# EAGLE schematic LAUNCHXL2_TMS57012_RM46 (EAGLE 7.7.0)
DOC_NUMBER: LAUNCHXL2_TMS57012_RM46; REV: B

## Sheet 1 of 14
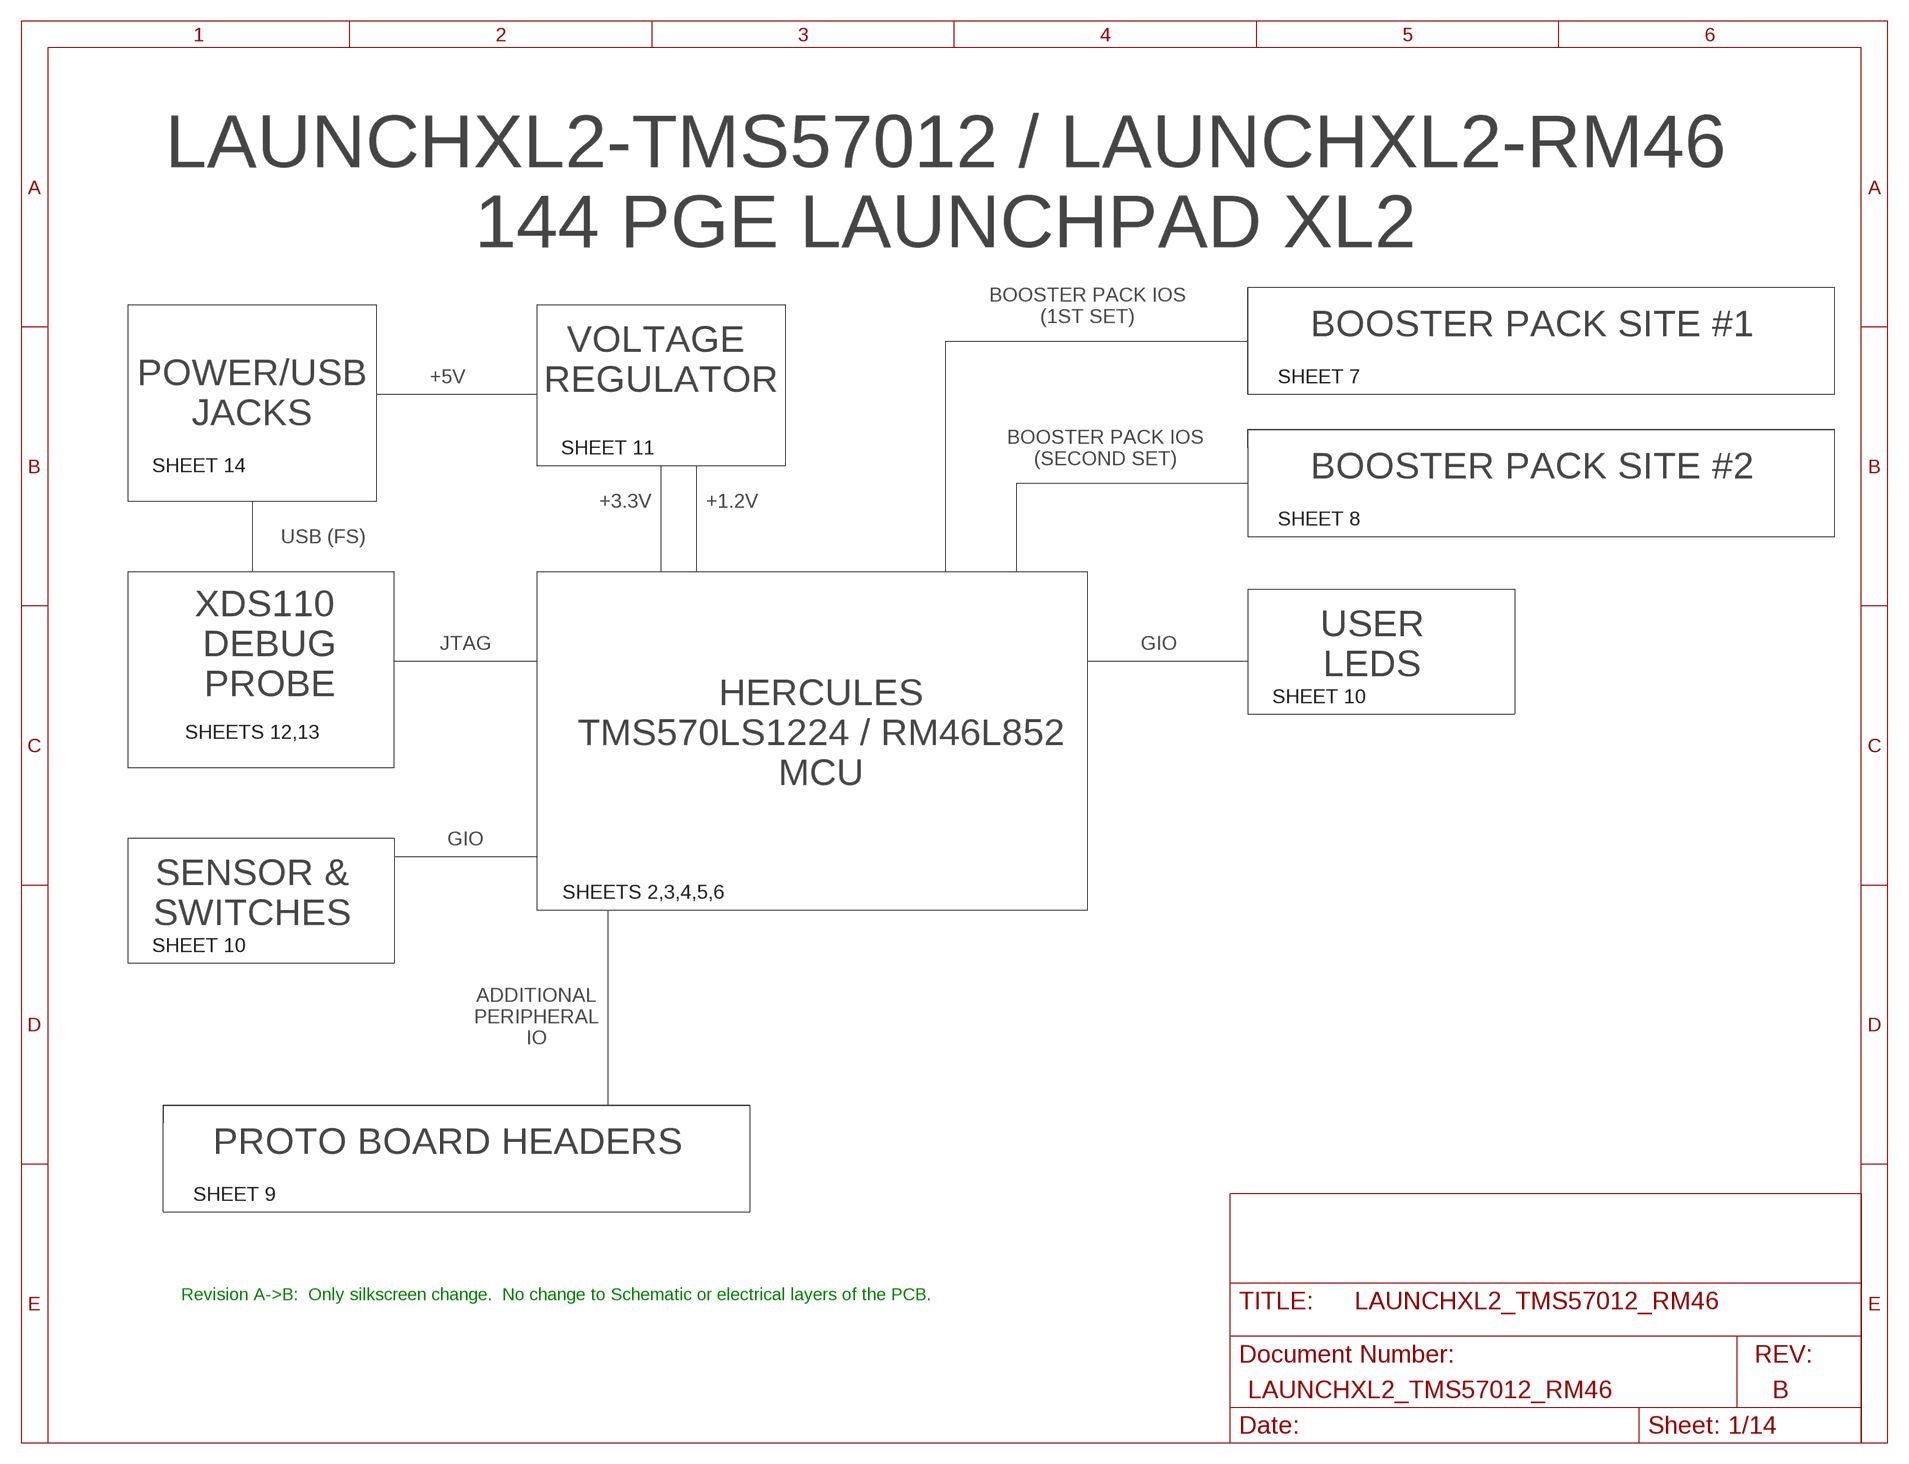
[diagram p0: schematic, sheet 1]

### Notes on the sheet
- LAUNCHXL2-TMS57012 / LAUNCHXL2-RM46
  144 PGE LAUNCHPAD XL2
- BOOSTER PACK IOS
  (1ST SET)
- BOOSTER PACK SITE #1
- VOLTAGE 
  REGULATOR
- +5V | SHEET 7
- POWER/USB
  JACKS
- SHEET 11
- BOOSTER PACK IOS
  (SECOND SET)
- SHEET 14 | BOOSTER PACK SITE #2
- +3.3V | +1.2V
- SHEET 8
- USB (FS)
- XDS110 
  DEBUG
  PROBE
- JTAG | GIO
- USER
  LEDS
- SHEET 10
- SHEETS 12,13
- HERCULES
  TMS570LS1224 / RM46L852
  MCU
- GIO
- SENSOR &
  SWITCHES
- SHEETS 2,3,4,5,6
- SHEET 10
- ADDITIONAL
  PERIPHERAL
  IO
- PROTO BOARD HEADERS
- SHEET 9
- Revision A->B:  Only silkscreen change.  No change to Schematic or electrical layers of the PCB.

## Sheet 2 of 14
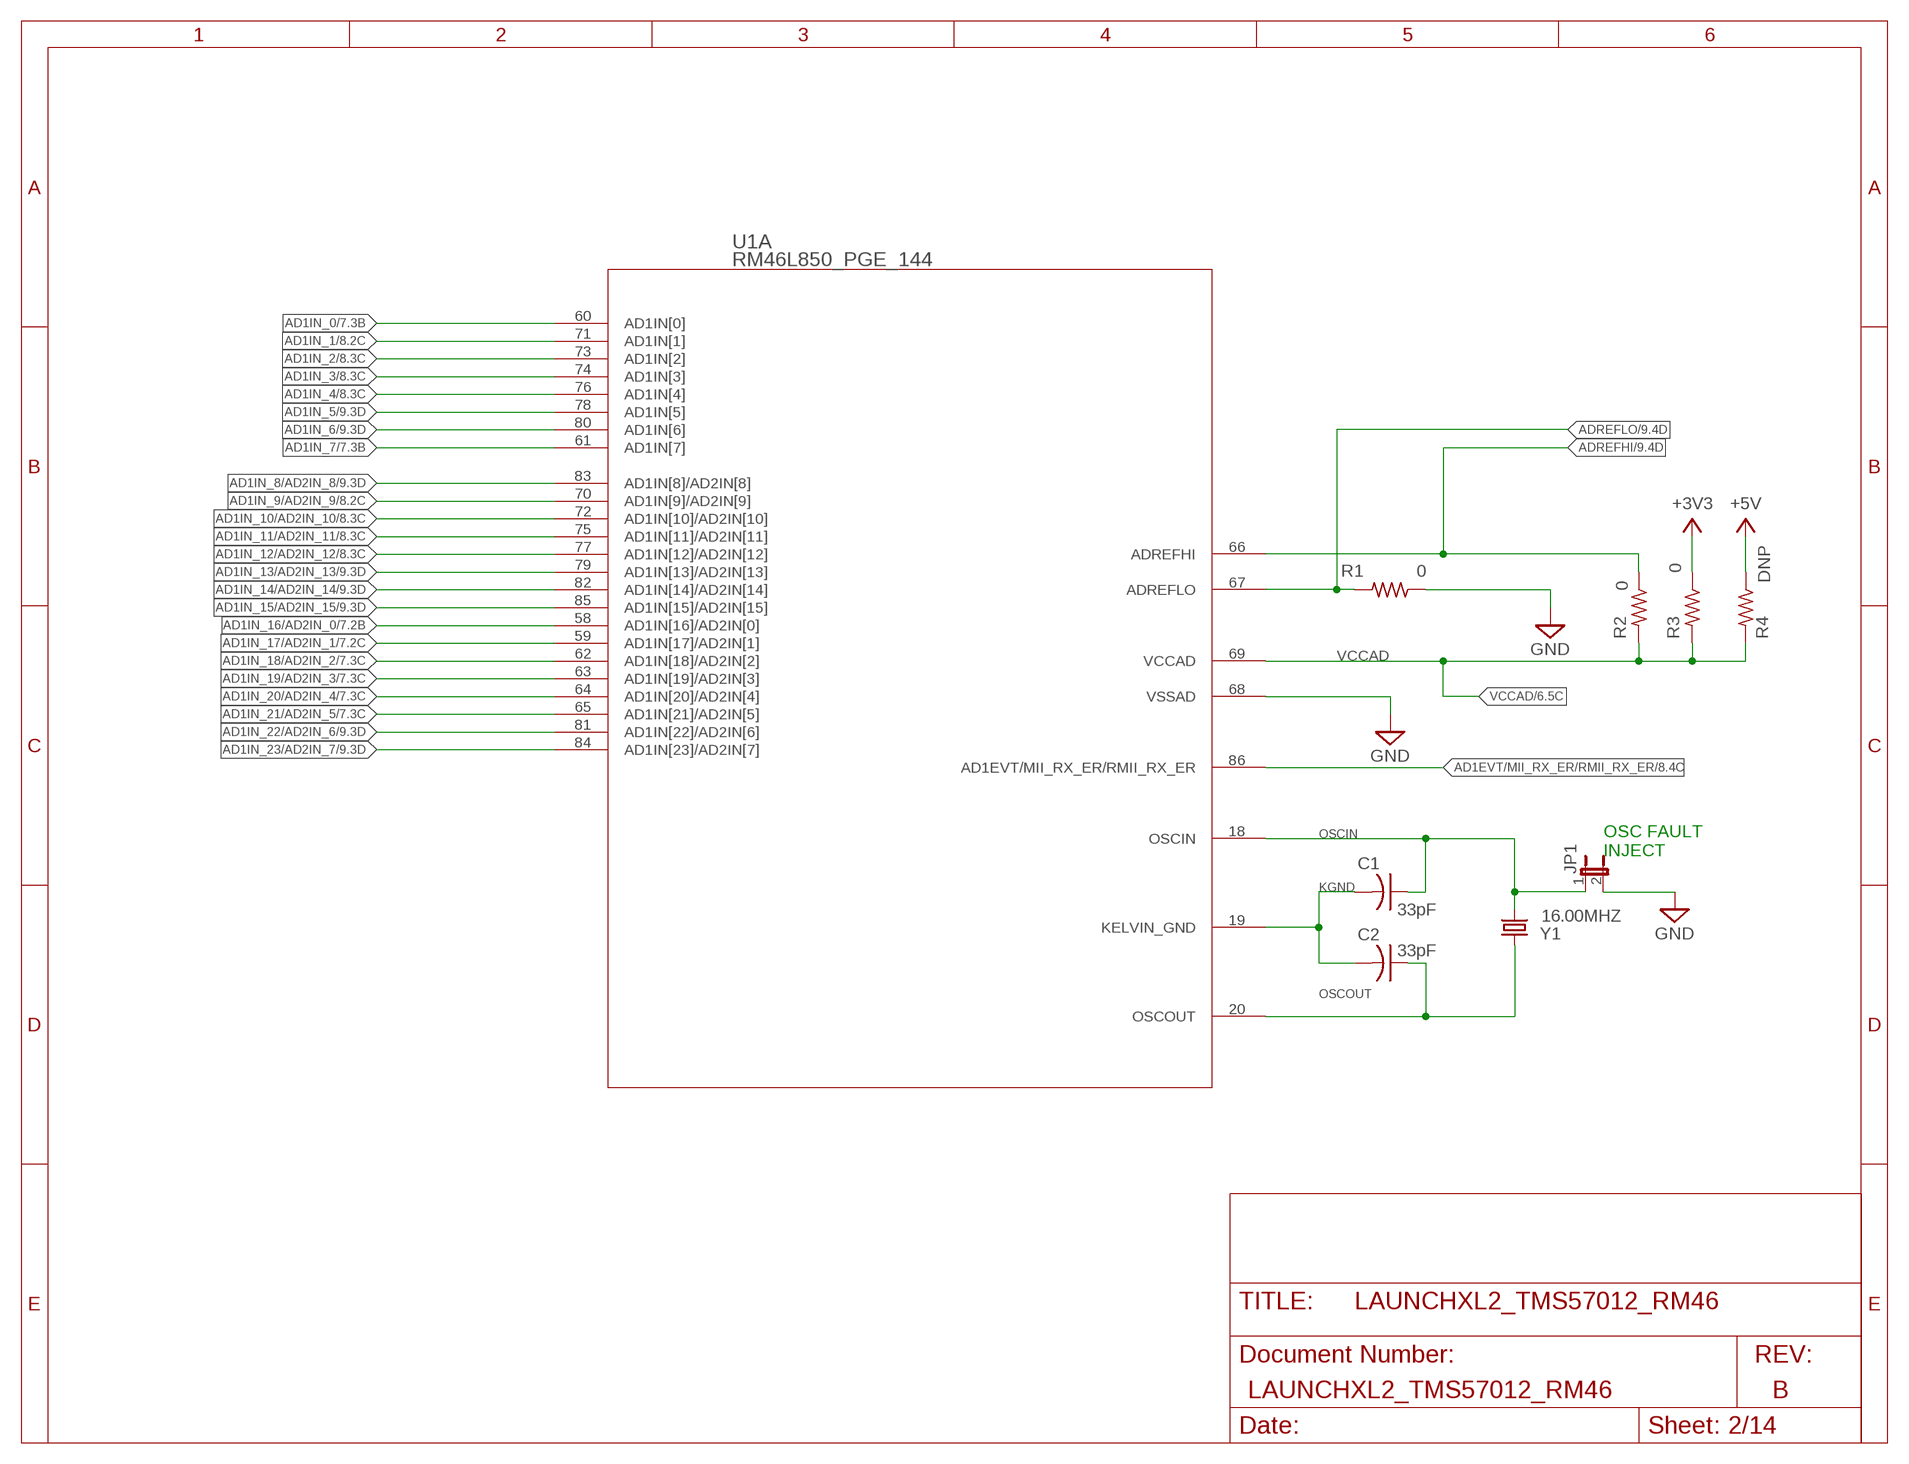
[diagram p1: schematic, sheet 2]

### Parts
C1  33pF  C-USC0402K  [C0402K]
C2  33pF  C-USC0402K  [C0402K]
JP1  SHUNT_HANG_OFF  JP1E  [JP1]
R1  0  R-US_R0402  [R0402]
R2  0  R-US_R0402  [R0402]
R3  0  R-US_R0402  [R0402]
R4  DNP  R-US_R0402  [R0402]
U1  RM46L850_PGE_144  [PGE144]
Y1  16.00MHZ  CRYSTAL  [ABLS]

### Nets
+3V3: R3.1 ; also sheet 3,5,6,7,8,9,10,11,12,13
+5V: R4.1 ; also sheet 7,8,9,11,14
AD1EVT/MII_RX_ER/RMII_RX_ER: U1.86(A:AD1EVT/MII_RX_ER/RMII_RX_ER) ; also sheet 8,9
AD1IN_0: U1.60(A:AD1IN[0]) ; also sheet 7
AD1IN_1: U1.71(A:AD1IN[1]) ; also sheet 8
AD1IN_2: U1.73(A:AD1IN[2]) ; also sheet 8
AD1IN_3: U1.74(A:AD1IN[3]) ; also sheet 8
AD1IN_4: U1.76(A:AD1IN[4]) ; also sheet 8
AD1IN_5: U1.78(A:AD1IN[5]) ; also sheet 9
AD1IN_6: U1.80(A:AD1IN[6]) ; also sheet 9,10
AD1IN_7: U1.61(A:AD1IN[7]) ; also sheet 7
AD1IN_8/AD2IN_8: U1.83(A:AD1IN[8]/AD2IN[8]) ; also sheet 9
AD1IN_9/AD2IN_9: U1.70(A:AD1IN[9]/AD2IN[9]) ; also sheet 8,9
AD1IN_10/AD2IN_10: U1.72(A:AD1IN[10]/AD2IN[10]) ; also sheet 8,9
AD1IN_11/AD2IN_11: U1.75(A:AD1IN[11]/AD2IN[11]) ; also sheet 8,9
AD1IN_12/AD2IN_12: U1.77(A:AD1IN[12]/AD2IN[12]) ; also sheet 8,9
AD1IN_13/AD2IN_13: U1.79(A:AD1IN[13]/AD2IN[13]) ; also sheet 9
AD1IN_14/AD2IN_14: U1.82(A:AD1IN[14]/AD2IN[14]) ; also sheet 9
AD1IN_15/AD2IN_15: U1.85(A:AD1IN[15]/AD2IN[15]) ; also sheet 9
AD1IN_16/AD2IN_0: U1.58(A:AD1IN[16]/AD2IN[0]) ; also sheet 7,9
AD1IN_17/AD2IN_1: U1.59(A:AD1IN[17]/AD2IN[1]) ; also sheet 7,9
AD1IN_18/AD2IN_2: U1.62(A:AD1IN[18]/AD2IN[2]) ; also sheet 7,9
AD1IN_19/AD2IN_3: U1.63(A:AD1IN[19]/AD2IN[3]) ; also sheet 7,9
AD1IN_20/AD2IN_4: U1.64(A:AD1IN[20]/AD2IN[4]) ; also sheet 7,9
AD1IN_21/AD2IN_5: U1.65(A:AD1IN[21]/AD2IN[5]) ; also sheet 7,9
AD1IN_22/AD2IN_6: U1.81(A:AD1IN[22]/AD2IN[6]) ; also sheet 9
AD1IN_23/AD2IN_7: U1.84(A:AD1IN[23]/AD2IN[7]) ; also sheet 9
ADREFHI: R2.1 U1.66(A:ADREFHI) ; also sheet 9
ADREFLO: R1.2 U1.67(A:ADREFLO) ; also sheet 9
GND: JP1.2 R1.1 U1.68(A:VSSAD) ; also sheet 3,5,6,7,8,9,10,11,12,13,14
KGND: C1.2 C2.2 U1.19(A:KELVIN_GND)
OSCIN: C1.1 JP1.1 U1.18(A:OSCIN) Y1.2
OSCOUT: C2.1 U1.20(A:OSCOUT) Y1.1
VCCAD: R2.2 R3.2 R4.2 U1.69(A:VCCAD) ; also sheet 6

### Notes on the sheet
- OSC FAULT
  INJECT

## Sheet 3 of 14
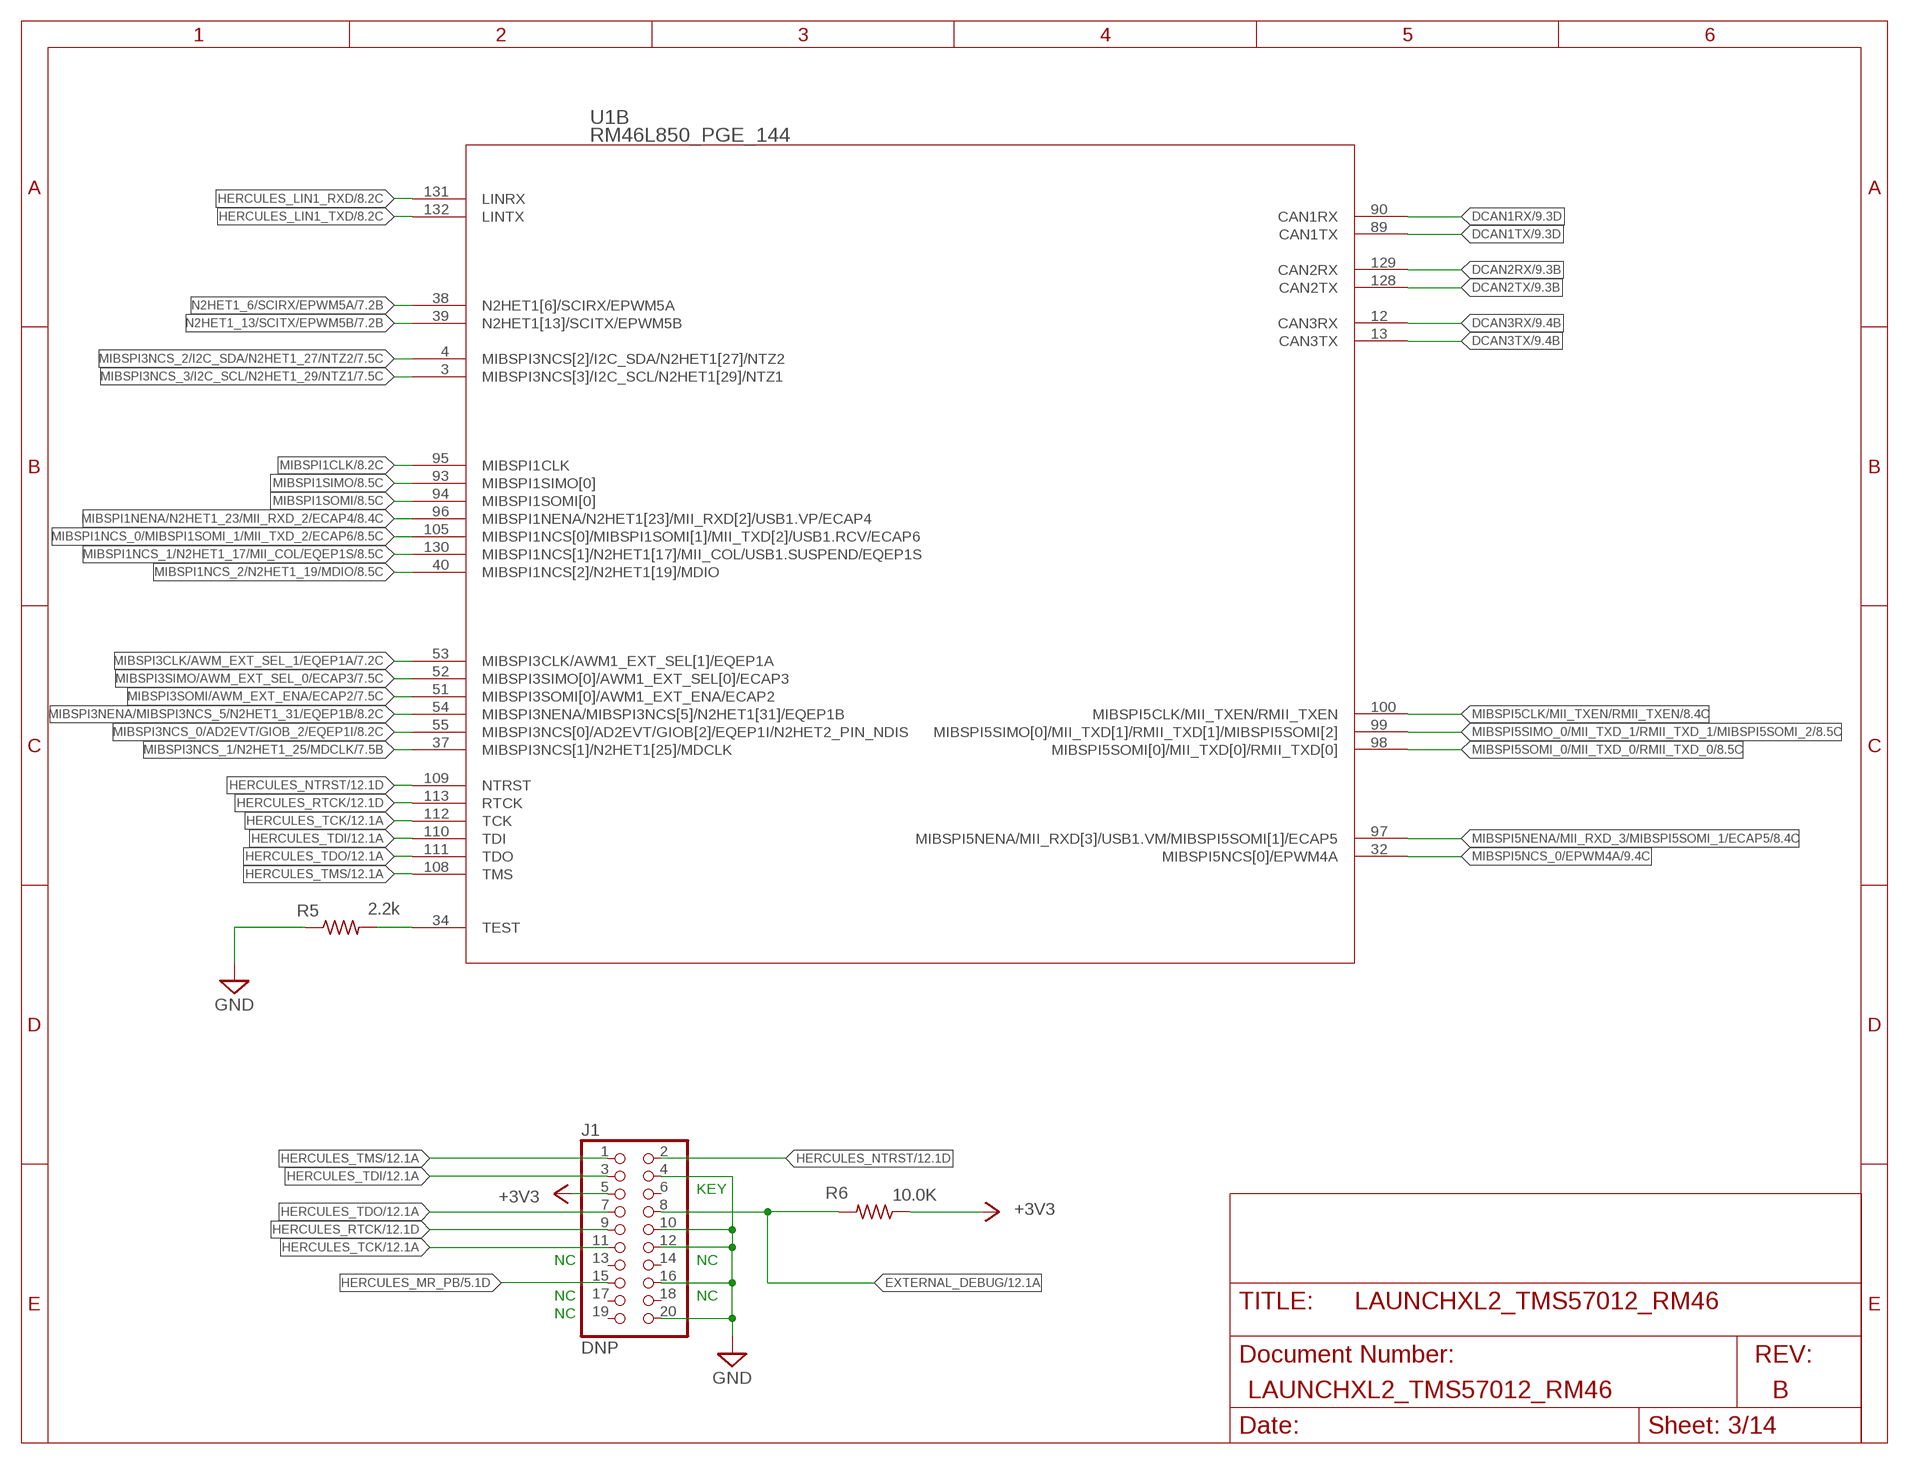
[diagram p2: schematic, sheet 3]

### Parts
J1  DNP  PINHD-2X10SAMTEC-FTR-110-51-S-D-06  [SAMTEC-FTR-110-51-S-D-06]
R5  2.2k  R-US_R0402  [R0402]
R6  10.0K  R-US_R0402  [R0402]

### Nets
+3V3: J1.5 R6.1 ; also sheet 2,5,6,7,8,9,10,11,12,13
DCAN1RX: U1.90(B:CAN1RX) ; also sheet 9
DCAN1TX: U1.89(B:CAN1TX) ; also sheet 9
DCAN2RX: U1.129(B:CAN2RX) ; also sheet 9
DCAN2TX: U1.128(B:CAN2TX) ; also sheet 9
DCAN3RX: U1.12(B:CAN3RX) ; also sheet 9
DCAN3TX: U1.13(B:CAN3TX) ; also sheet 9
EXTERNAL_DEBUG: J1.8 R6.2 ; also sheet 12
GND: J1.4 J1.10 J1.12 J1.16 J1.20 R5.1 ; also sheet 2,5,6,7,8,9,10,11,12,13,14
HERCULES_LIN1_RXD: U1.131(B:LINRX) ; also sheet 8,9,12
HERCULES_LIN1_TXD: U1.132(B:LINTX) ; also sheet 8,9,12
HERCULES_MR_PB: J1.15 ; also sheet 5,12
HERCULES_NTRST: J1.2 U1.109(B:NTRST) ; also sheet 12
HERCULES_RTCK: J1.9 U1.113(B:RTCK) ; also sheet 12
HERCULES_TCK: J1.11 U1.112(B:TCK) ; also sheet 12
HERCULES_TDI: J1.3 U1.110(B:TDI) ; also sheet 12
HERCULES_TDO: J1.7 U1.111(B:TDO) ; also sheet 12
HERCULES_TMS: J1.1 U1.108(B:TMS) ; also sheet 12
MIBSPI1CLK: U1.95(B:MIBSPI1CLK) ; also sheet 8,9
MIBSPI1NCS_0/MIBSPI1SOMI_1/MII_TXD_2/ECAP6: U1.105(B:MIBSPI1NCS[0]/MIBSPI1SOMI[1]/MII_TXD[2]/USB1.RCV/ECAP6) ; also sheet 8,9
MIBSPI1NCS_1/N2HET1_17/MII_COL/EQEP1S: U1.130(B:MIBSPI1NCS[1]/N2HET1[17]/MII_COL/USB1.SUSPEND/EQEP1S) ; also sheet 8,9
MIBSPI1NCS_2/N2HET1_19/MDIO: U1.40(B:MIBSPI1NCS[2]/N2HET1[19]/MDIO) ; also sheet 8,9
MIBSPI1NENA/N2HET1_23/MII_RXD_2/ECAP4: U1.96(B:MIBSPI1NENA/N2HET1[23]/MII_RXD[2]/USB1.VP/ECAP4) ; also sheet 8,9
MIBSPI1SIMO: U1.93(B:MIBSPI1SIMO[0]) ; also sheet 8,9
MIBSPI1SOMI: U1.94(B:MIBSPI1SOMI[0]) ; also sheet 8,9
MIBSPI3CLK/AWM_EXT_SEL_1/EQEP1A: U1.53(B:MIBSPI3CLK/AWM1_EXT_SEL[1]/EQEP1A) ; also sheet 7,9
MIBSPI3NCS_0/AD2EVT/GIOB_2/EQEP1I: U1.55(B:MIBSPI3NCS[0]/AD2EVT/GIOB[2]/EQEP1I/N2HET2_PIN_NDIS) ; also sheet 8,9,10
MIBSPI3NCS_1/N2HET1_25/MDCLK: U1.37(B:MIBSPI3NCS[1]/N2HET1[25]/MDCLK) ; also sheet 7,9
MIBSPI3NCS_2/I2C_SDA/N2HET1_27/NTZ2: U1.4(B:MIBSPI3NCS[2]/I2C_SDA/N2HET1[27]/NTZ2) ; also sheet 7,9
MIBSPI3NCS_3/I2C_SCL/N2HET1_29/NTZ1: U1.3(B:MIBSPI3NCS[3]/I2C_SCL/N2HET1[29]/NTZ1) ; also sheet 7,9
MIBSPI3NENA/MIBSPI3NCS_5/N2HET1_31/EQEP1B: U1.54(B:MIBSPI3NENA/MIBSPI3NCS[5]/N2HET1[31]/EQEP1B) ; also sheet 8,9
MIBSPI3SIMO/AWM_EXT_SEL_0/ECAP3: U1.52(B:MIBSPI3SIMO[0]/AWM1_EXT_SEL[0]/ECAP3) ; also sheet 7,9
MIBSPI3SOMI/AWM_EXT_ENA/ECAP2: U1.51(B:MIBSPI3SOMI[0]/AWM1_EXT_ENA/ECAP2) ; also sheet 7,9
MIBSPI5CLK/MII_TXEN/RMII_TXEN: U1.100(B:MIBSPI5CLK/MII_TXEN/RMII_TXEN) ; also sheet 8,9
MIBSPI5NCS_0/EPWM4A: U1.32(B:MIBSPI5NCS[0]/EPWM4A) ; also sheet 9
MIBSPI5NENA/MII_RXD_3/MIBSPI5SOMI_1/ECAP5: U1.97(B:MIBSPI5NENA/MII_RXD[3]/USB1.VM/MIBSPI5SOMI[1]/ECAP5) ; also sheet 8,9
MIBSPI5SIMO_0/MII_TXD_1/RMII_TXD_1/MIBSPI5SOMI_2: U1.99(B:MIBSPI5SIMO[0]/MII_TXD[1]/RMII_TXD[1]/MIBSPI5SOMI[2]) ; also sheet 8,9
MIBSPI5SOMI_0/MII_TXD_0/RMII_TXD_0: U1.98(B:MIBSPI5SOMI[0]/MII_TXD[0]/RMII_TXD[0]) ; also sheet 8,9
N2HET1_6/SCIRX/EPWM5A: U1.38(B:N2HET1[6]/SCIRX/EPWM5A) ; also sheet 7,9
N2HET1_13/SCITX/EPWM5B: U1.39(B:N2HET1[13]/SCITX/EPWM5B) ; also sheet 7,9
N$39: R5.2 U1.34(B:TEST)
Unconnected: J1.6 J1.13 J1.14 J1.17 J1.18 J1.19

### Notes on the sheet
- KEY
- NC | NC
- NC | NC
- NC

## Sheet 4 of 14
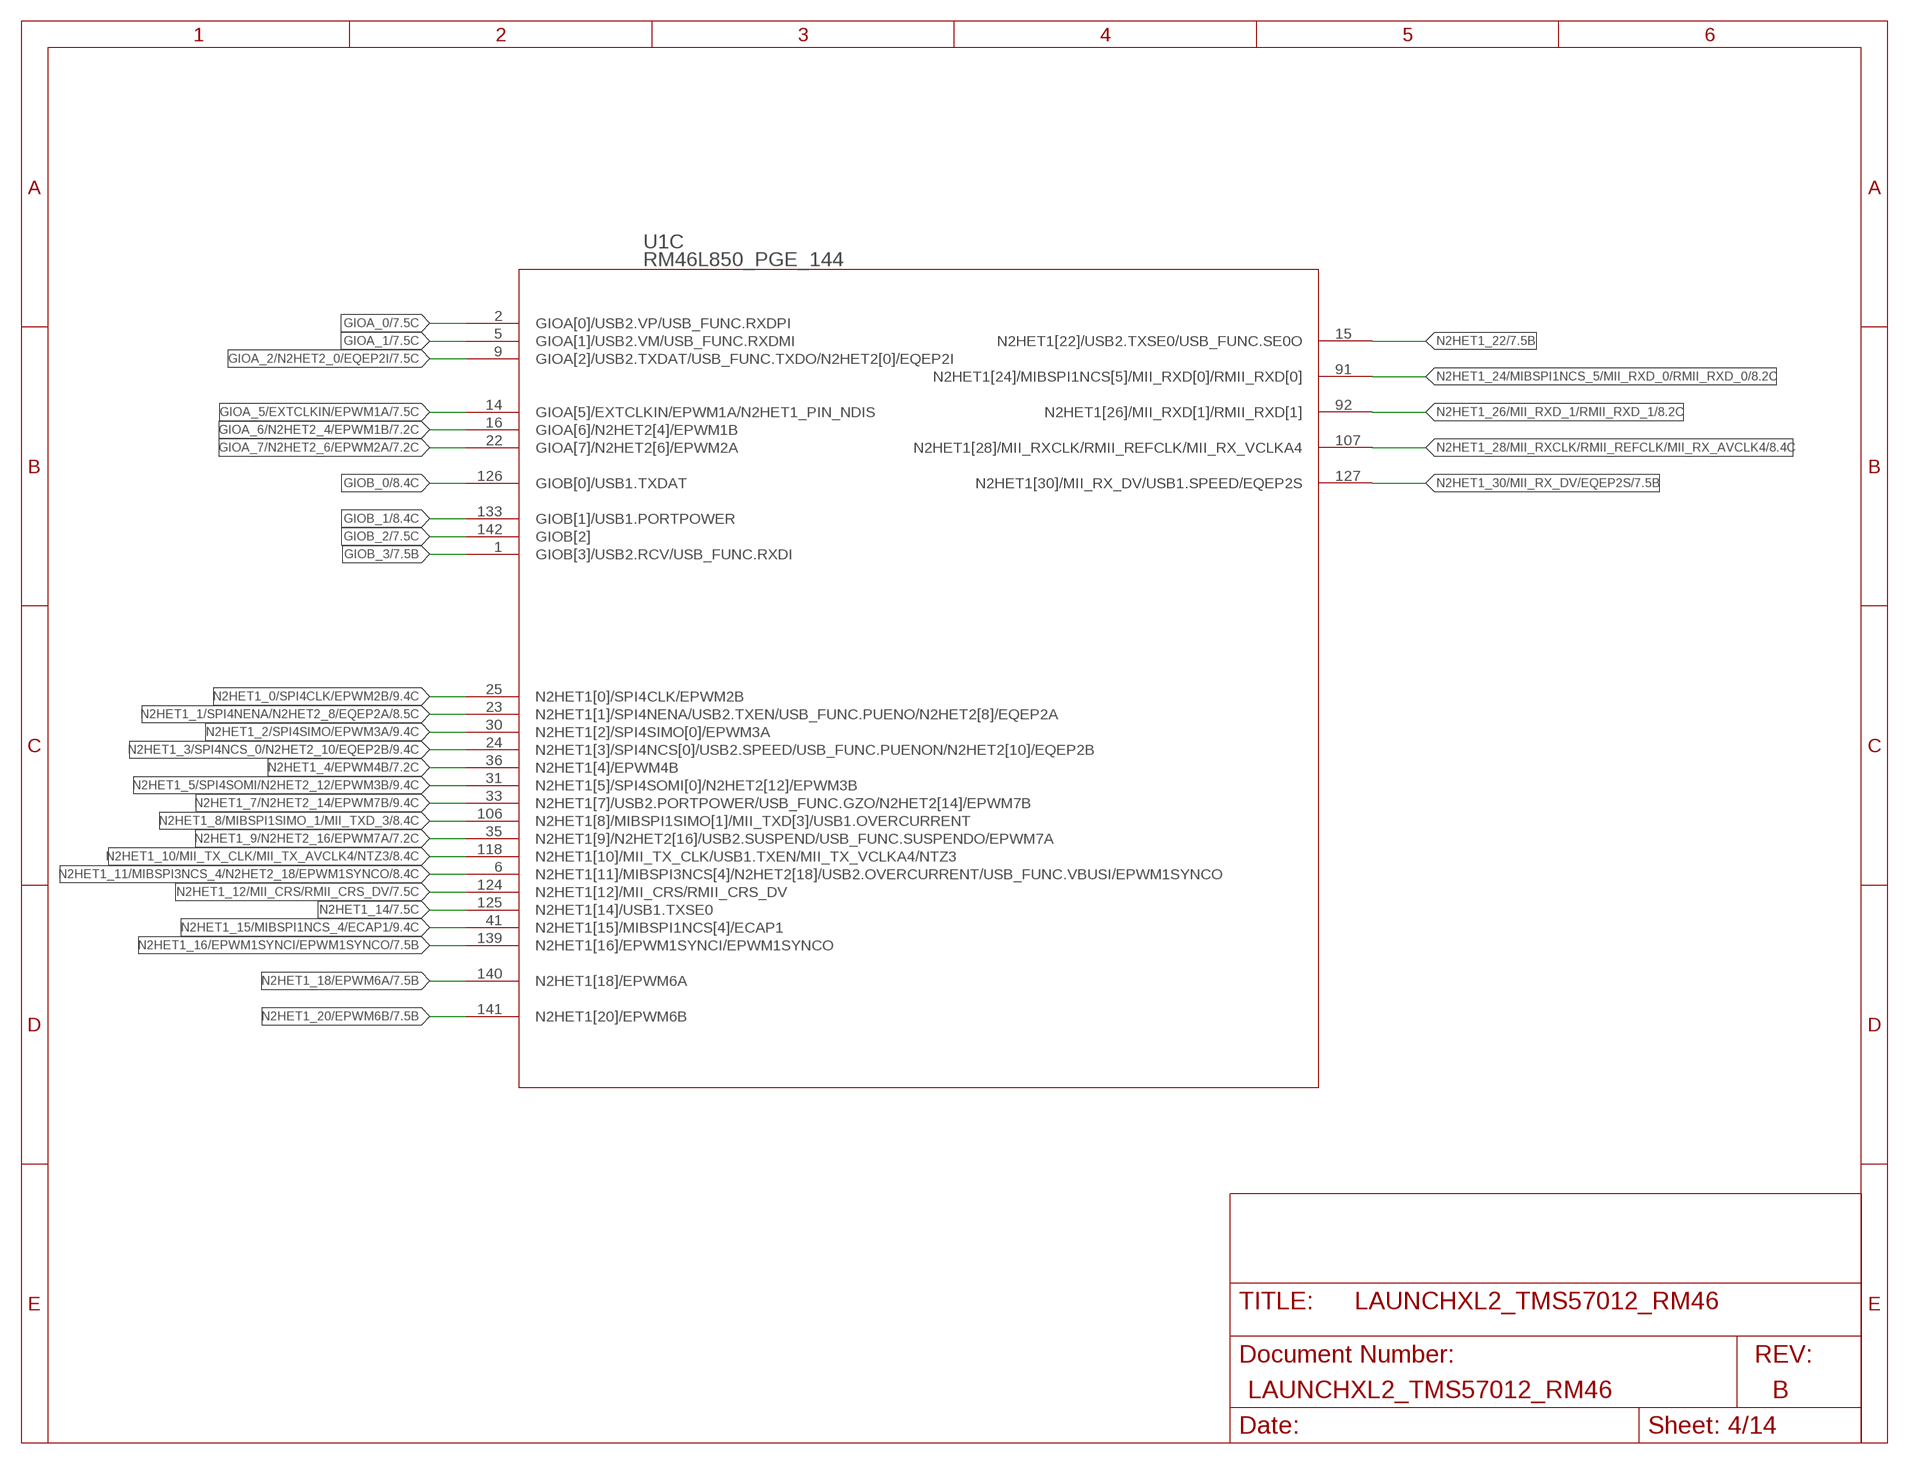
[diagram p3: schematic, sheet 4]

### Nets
GIOA_0: U1.2(C:GIOA[0]/USB2.VP/USB_FUNC.RXDPI) ; also sheet 7,9
GIOA_1: U1.5(C:GIOA[1]/USB2.VM/USB_FUNC.RXDMI) ; also sheet 7,9
GIOA_2/N2HET2_0/EQEP2I: U1.9(C:GIOA[2]/USB2.TXDAT/USB_FUNC.TXDO/N2HET2[0]/EQEP2I) ; also sheet 7,9
GIOA_5/EXTCLKIN/EPWM1A: U1.14(C:GIOA[5]/EXTCLKIN/EPWM1A/N2HET1_PIN_NDIS) ; also sheet 7,9
GIOA_6/N2HET2_4/EPWM1B: U1.16(C:GIOA[6]/N2HET2[4]/EPWM1B) ; also sheet 7,9
GIOA_7/N2HET2_6/EPWM2A: U1.22(C:GIOA[7]/N2HET2[6]/EPWM2A) ; also sheet 7,9
GIOB_0: U1.126(C:GIOB[0]/USB1.TXDAT) ; also sheet 8,9
GIOB_1: U1.133(C:GIOB[1]/USB1.PORTPOWER) ; also sheet 8,9,10
GIOB_2: U1.142(C:GIOB[2]) ; also sheet 7,9,10
GIOB_3: U1.1(C:GIOB[3]/USB2.RCV/USB_FUNC.RXDI) ; also sheet 7,9
N2HET1_0/SPI4CLK/EPWM2B: U1.25(C:N2HET1[0]/SPI4CLK/EPWM2B) ; also sheet 9
N2HET1_1/SPI4NENA/N2HET2_8/EQEP2A: U1.23(C:N2HET1[1]/SPI4NENA/USB2.TXEN/USB_FUNC.PUENO/N2HET2[8]/EQEP2A) ; also sheet 8,9
N2HET1_2/SPI4SIMO/EPWM3A: U1.30(C:N2HET1[2]/SPI4SIMO[0]/EPWM3A) ; also sheet 9
N2HET1_3/SPI4NCS_0/N2HET2_10/EQEP2B: U1.24(C:N2HET1[3]/SPI4NCS[0]/USB2.SPEED/USB_FUNC.PUENON/N2HET2[10]/EQEP2B) ; also sheet 9
N2HET1_4/EPWM4B: U1.36(C:N2HET1[4]/EPWM4B) ; also sheet 7,9
N2HET1_5/SPI4SOMI/N2HET2_12/EPWM3B: U1.31(C:N2HET1[5]/SPI4SOMI[0]/N2HET2[12]/EPWM3B) ; also sheet 9
N2HET1_7/N2HET2_14/EPWM7B: U1.33(C:N2HET1[7]/USB2.PORTPOWER/USB_FUNC.GZO/N2HET2[14]/EPWM7B) ; also sheet 9
N2HET1_8/MIBSPI1SIMO_1/MII_TXD_3: U1.106(C:N2HET1[8]/MIBSPI1SIMO[1]/MII_TXD[3]/USB1.OVERCURRENT) ; also sheet 8,9
N2HET1_9/N2HET2_16/EPWM7A: U1.35(C:N2HET1[9]/N2HET2[16]/USB2.SUSPEND/USB_FUNC.SUSPENDO/EPWM7A) ; also sheet 7,9
N2HET1_10/MII_TX_CLK/MII_TX_AVCLK4/NTZ3: U1.118(C:N2HET1[10]/MII_TX_CLK/USB1.TXEN/MII_TX_VCLKA4/NTZ3) ; also sheet 8,9
N2HET1_11/MIBSPI3NCS_4/N2HET2_18/EPWM1SYNCO: U1.6(C:N2HET1[11]/MIBSPI3NCS[4]/N2HET2[18]/USB2.OVERCURRENT/USB_FUNC.VBUSI/EPWM1SYNCO) ; also sheet 8,9
N2HET1_12/MII_CRS/RMII_CRS_DV: U1.124(C:N2HET1[12]/MII_CRS/RMII_CRS_DV) ; also sheet 7,9
N2HET1_14: U1.125(C:N2HET1[14]/USB1.TXSE0) ; also sheet 7,9
N2HET1_15/MIBSPI1NCS_4/ECAP1: U1.41(C:N2HET1[15]/MIBSPI1NCS[4]/ECAP1) ; also sheet 9,10
N2HET1_16/EPWM1SYNCI/EPWM1SYNCO: U1.139(C:N2HET1[16]/EPWM1SYNCI/EPWM1SYNCO) ; also sheet 7,9
N2HET1_18/EPWM6A: U1.140(C:N2HET1[18]/EPWM6A) ; also sheet 7,9
N2HET1_20/EPWM6B: U1.141(C:N2HET1[20]/EPWM6B) ; also sheet 7,9
N2HET1_22: U1.15(C:N2HET1[22]/USB2.TXSE0/USB_FUNC.SE0O) ; also sheet 7,9
N2HET1_24/MIBSPI1NCS_5/MII_RXD_0/RMII_RXD_0: U1.91(C:N2HET1[24]/MIBSPI1NCS[5]/MII_RXD[0]/RMII_RXD[0]) ; also sheet 8,9
N2HET1_26/MII_RXD_1/RMII_RXD_1: U1.92(C:N2HET1[26]/MII_RXD[1]/RMII_RXD[1]) ; also sheet 8,9
N2HET1_28/MII_RXCLK/RMII_REFCLK/MII_RX_AVCLK4: U1.107(C:N2HET1[28]/MII_RXCLK/RMII_REFCLK/MII_RX_VCLKA4) ; also sheet 8,9
N2HET1_30/MII_RX_DV/EQEP2S: U1.127(C:N2HET1[30]/MII_RX_DV/USB1.SPEED/EQEP2S) ; also sheet 7,9

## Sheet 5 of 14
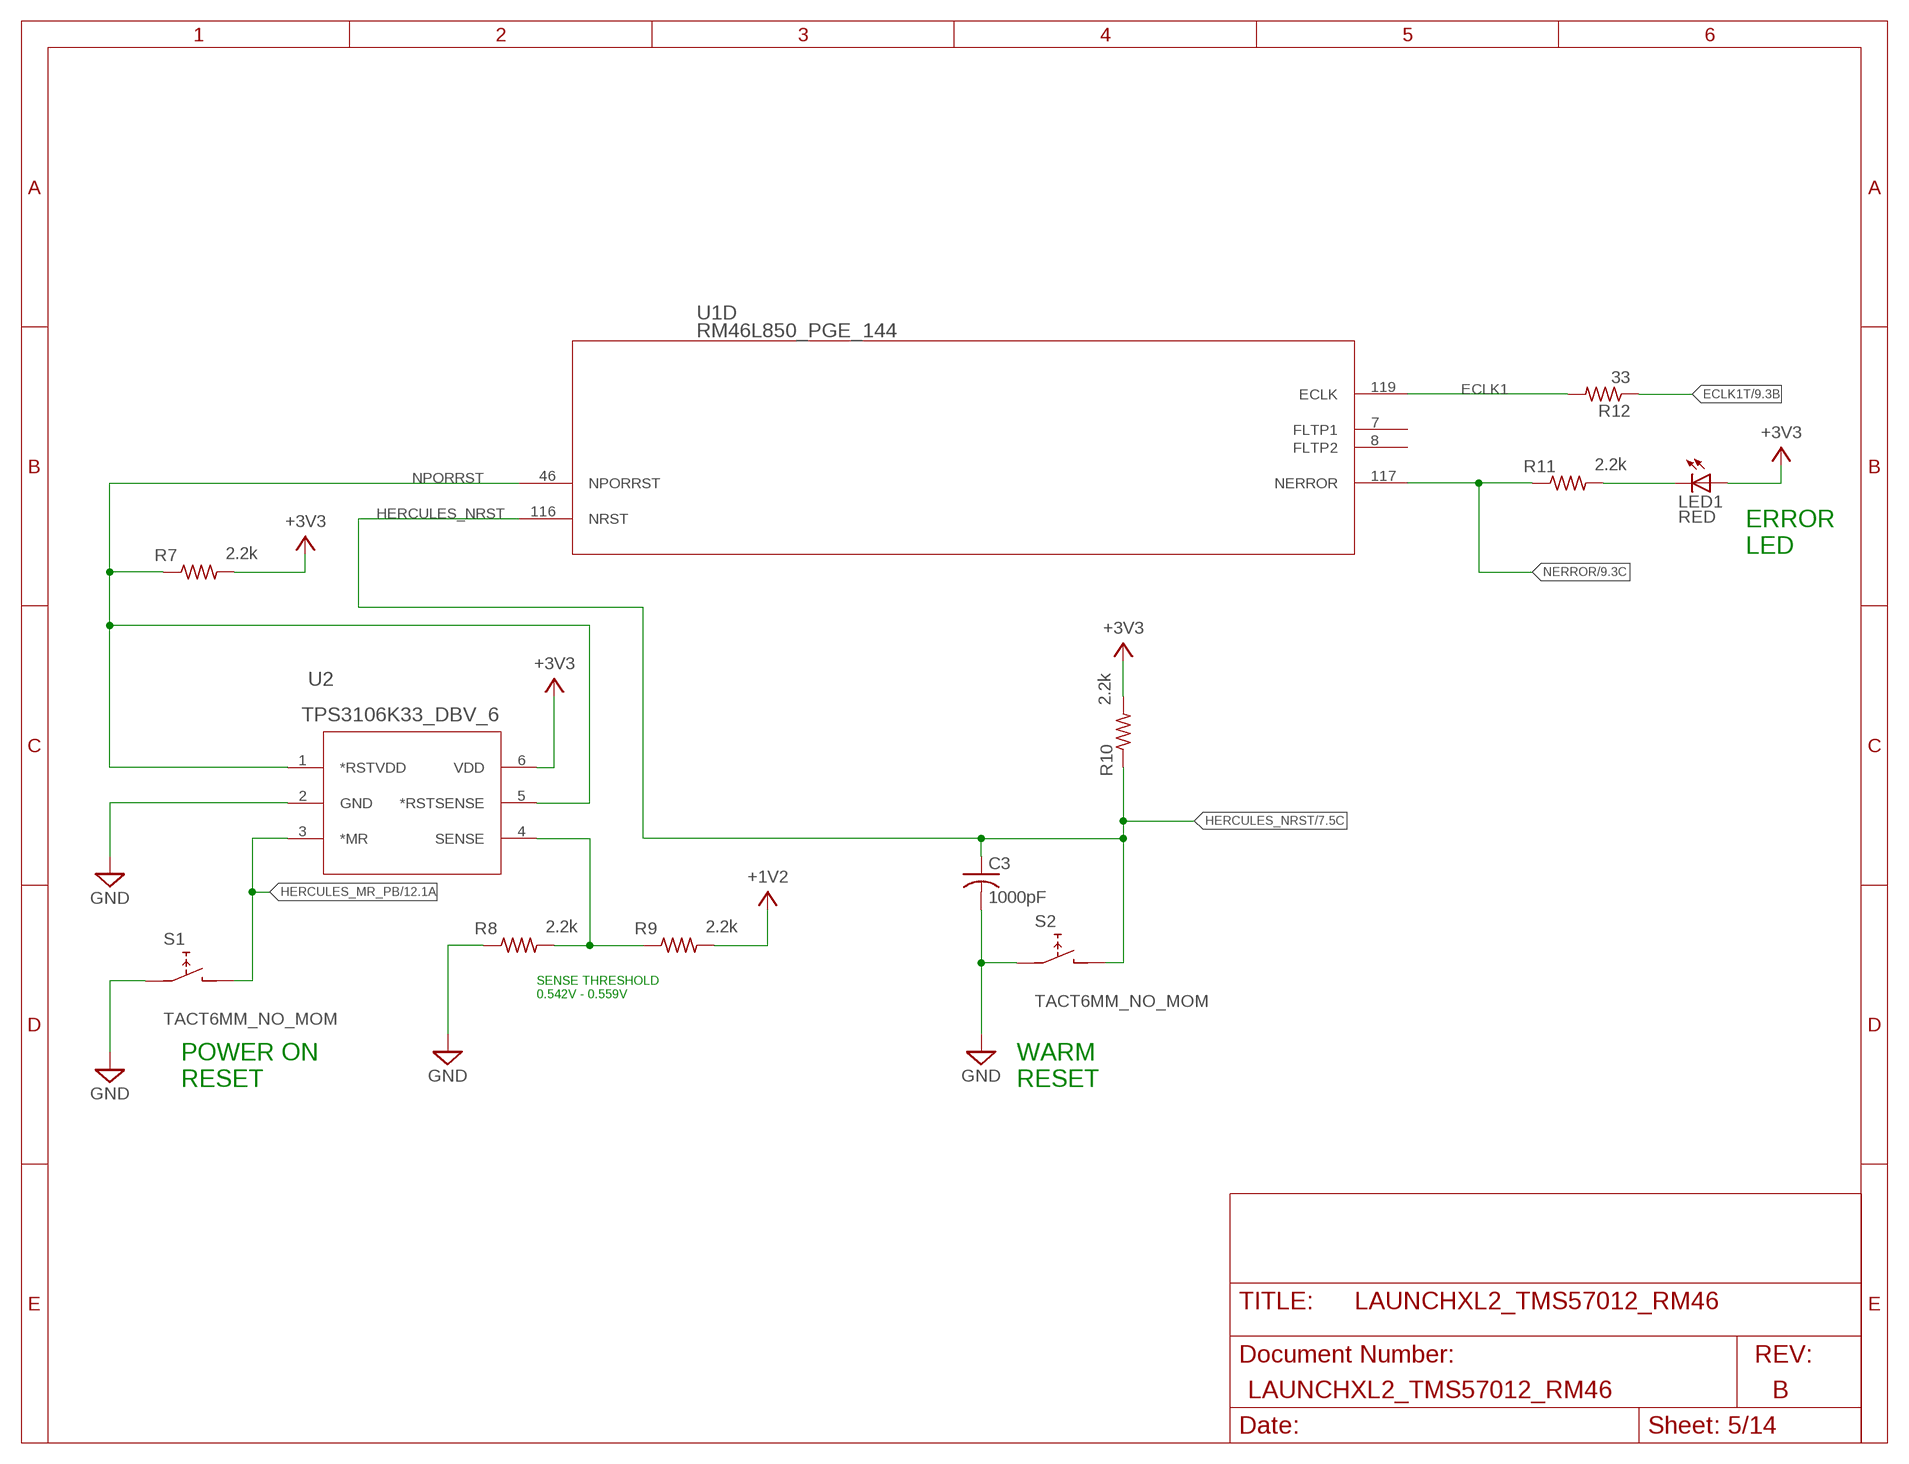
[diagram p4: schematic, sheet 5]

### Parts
C3  1000pF  C-USC0402  [C0402]
LED1  RED  LEDCHIPLED_0603  [CHIPLED_0603]
R7  2.2k  R-US_R0402  [R0402]
R8  2.2k  R-US_R0402  [R0402]
R9  2.2k  R-US_R0402  [R0402]
R10  2.2k  R-US_R0402  [R0402]
R11  2.2k  R-US_R0402  [R0402]
R12  33  R-US_R0402  [R0402]
S1  TACT6MM_NO_MOM  [CK_PTS645_SMD]
S2  TACT6MM_NO_MOM  [CK_PTS645_SMD]
U2  TPS3106K33_DBV_6  [DBV6]

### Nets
+1V2: R9.2 ; also sheet 6,11,12
+3V3: LED1.A R7.2 R10.2 U2.6(VDD) ; also sheet 2,3,6,7,8,9,10,11,12,13
ECLK1: R12.2 U1.119(D:ECLK)
ECLK1T: R12.1 ; also sheet 9
GND: C3.2 R8.1 S1.1 S1.2 S2.1 S2.2 U2.2(GND) ; also sheet 2,3,6,7,8,9,10,11,12,13,14
HERCULES_MR_PB: S1.3 S1.4 U2.3(*MR) ; also sheet 3,12
HERCULES_NRST: C3.1 R10.1 S2.3 S2.4 U1.116(D:NRST) ; also sheet 7,8,9,12
N$33: R8.2 R9.1 U2.4(SENSE)
N$34: LED1.C R11.2
NERROR: R11.1 U1.117(D:NERROR) ; also sheet 9
NPORRST: R7.1 U1.46(D:NPORRST) U2.1(*RSTVDD) U2.5(*RSTSENSE)
Unconnected: U1.7(D:FLTP1) U1.8(D:FLTP2)

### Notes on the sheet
- ERROR
  LED
- SENSE THRESHOLD 
  0.542V - 0.559V
- POWER ON
  RESET
- WARM
  RESET

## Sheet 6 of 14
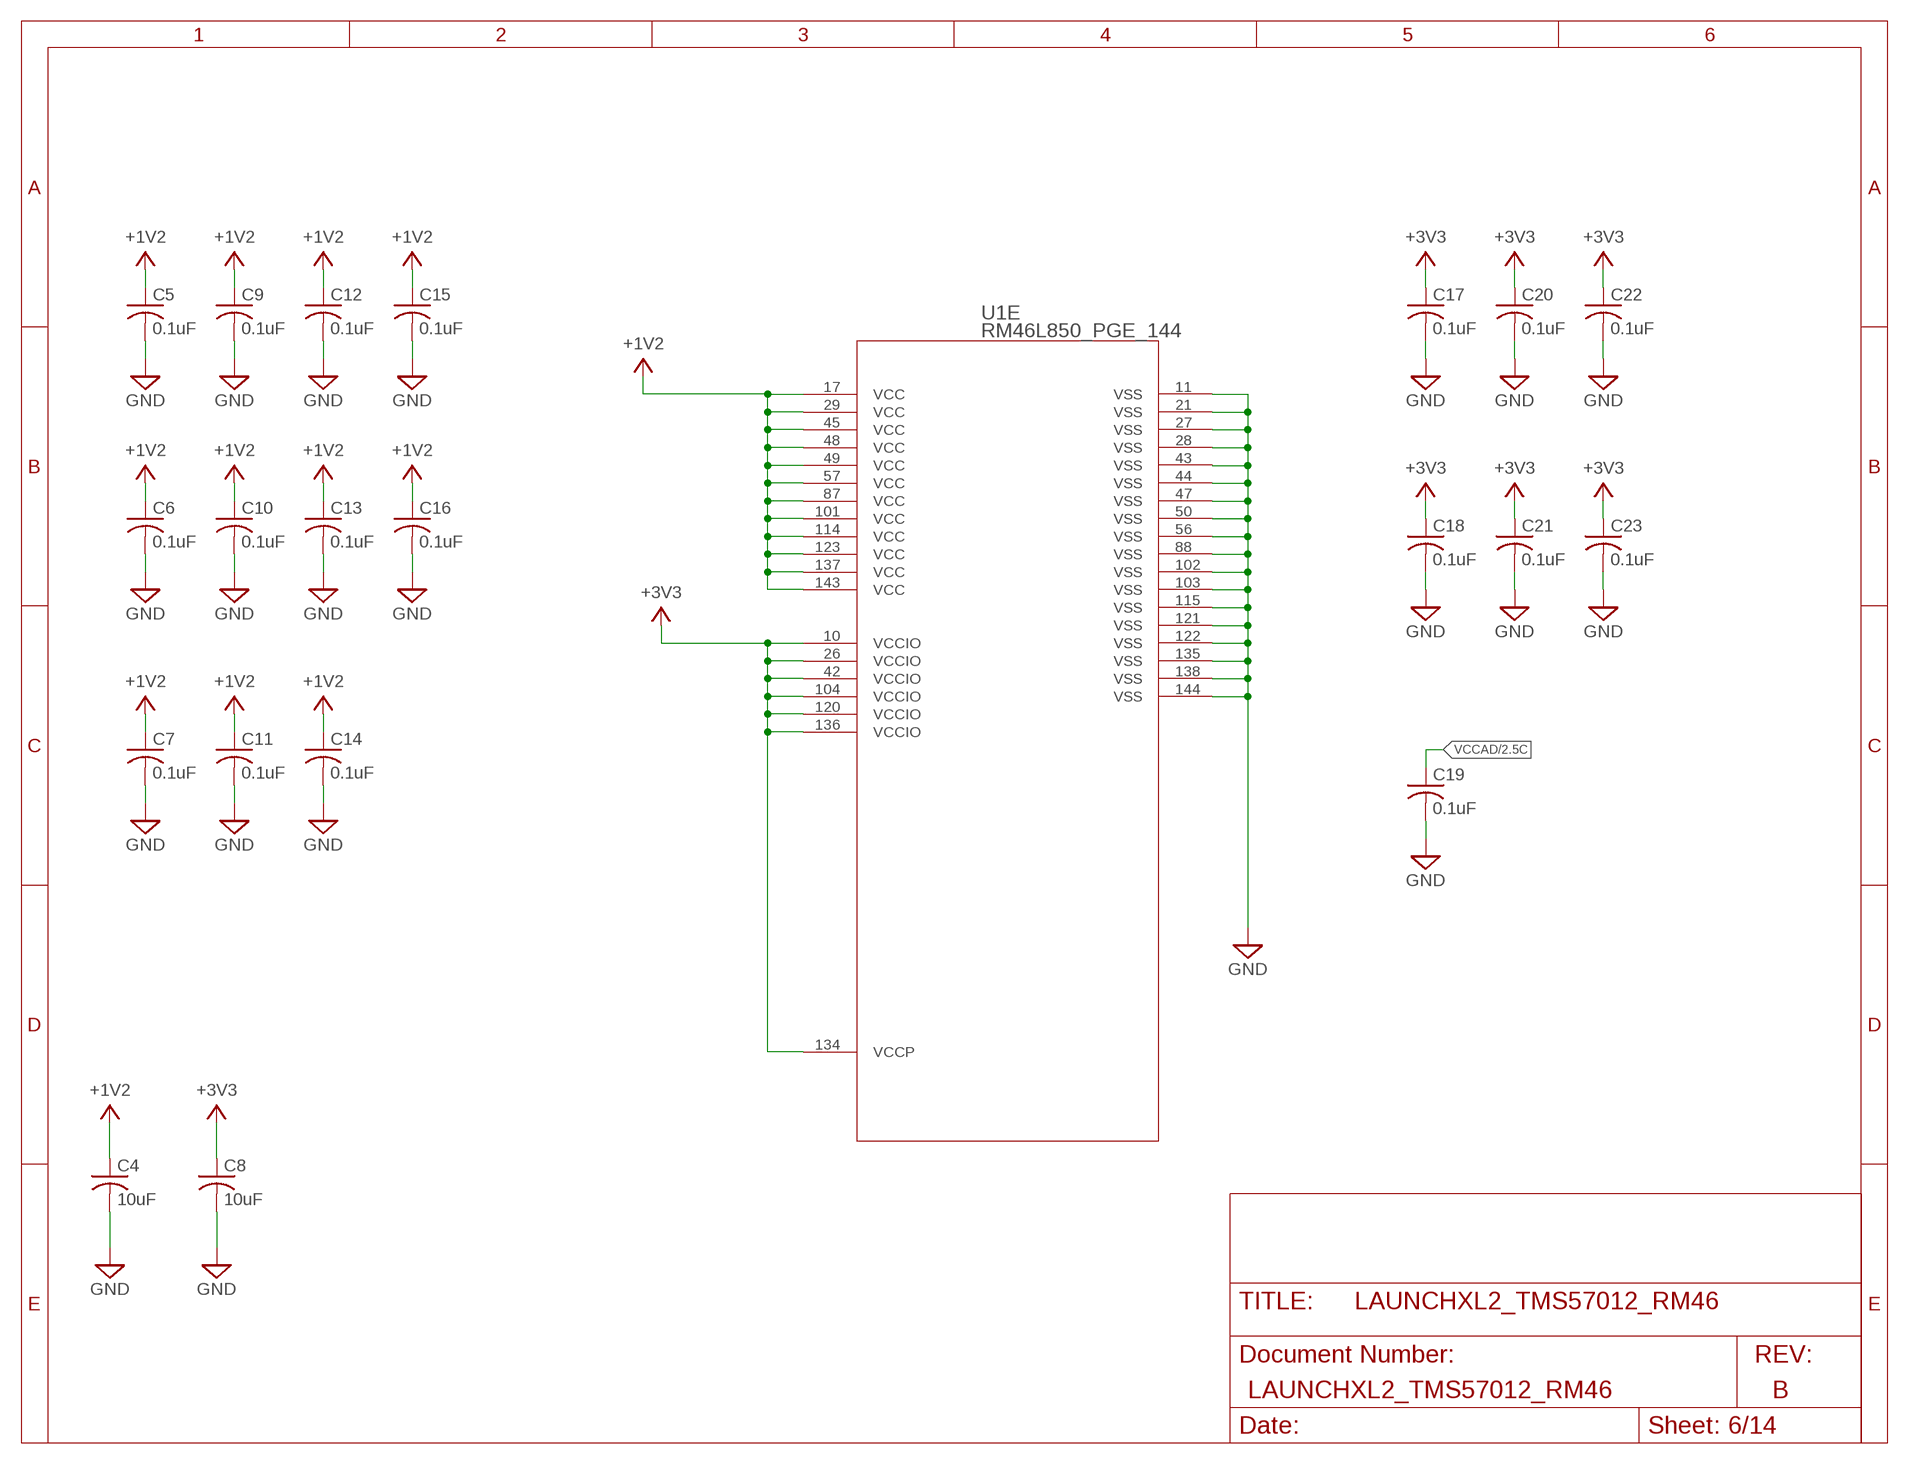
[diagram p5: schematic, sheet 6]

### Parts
C4  10uF  C-USC0805K  [C0805K]
C5  0.1uF  C-USC0402K  [C0402K]
C6  0.1uF  C-USC0402K  [C0402K]
C7  0.1uF  C-USC0402K  [C0402K]
C8  10uF  C-USC0805K  [C0805K]
C9  0.1uF  C-USC0402K  [C0402K]
C10  0.1uF  C-USC0402K  [C0402K]
C11  0.1uF  C-USC0402K  [C0402K]
C12  0.1uF  C-USC0402K  [C0402K]
C13  0.1uF  C-USC0402K  [C0402K]
C14  0.1uF  C-USC0402K  [C0402K]
C15  0.1uF  C-USC0402K  [C0402K]
C16  0.1uF  C-USC0402K  [C0402K]
C17  0.1uF  C-USC0402K  [C0402K]
C18  0.1uF  C-USC0402K  [C0402K]
C19  0.1uF  C-USC0402K  [C0402K]
C20  0.1uF  C-USC0402K  [C0402K]
C21  0.1uF  C-USC0402K  [C0402K]
C22  0.1uF  C-USC0402K  [C0402K]
C23  0.1uF  C-USC0402K  [C0402K]

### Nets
+1V2: C4.1 C5.1 C6.1 C7.1 C9.1 C10.1 C11.1 C12.1 C13.1 C14.1 C15.1 C16.1 U1.17(E:VCC) U1.29(E:VCC) U1.45(E:VCC) U1.48(E:VCC) U1.49(E:VCC) U1.57(E:VCC) U1.87(E:VCC) U1.101(E:VCC) U1.114(E:VCC) U1.123(E:VCC) U1.137(E:VCC) U1.143(E:VCC) ; also sheet 5,11,12
+3V3: C8.1 C17.1 C18.1 C20.1 C21.1 C22.1 C23.1 U1.10(E:VCCIO) U1.26(E:VCCIO) U1.42(E:VCCIO) U1.104(E:VCCIO) U1.120(E:VCCIO) U1.134(E:VCCP) U1.136(E:VCCIO) ; also sheet 2,3,5,7,8,9,10,11,12,13
GND: C4.2 C5.2 C6.2 C7.2 C8.2 C9.2 C10.2 C11.2 C12.2 C13.2 C14.2 C15.2 C16.2 C17.2 C18.2 C19.2 C20.2 C21.2 C22.2 C23.2 U1.11(E:VSS) U1.21(E:VSS) U1.27(E:VSS) U1.28(E:VSS) U1.43(E:VSS) U1.44(E:VSS) U1.47(E:VSS) U1.50(E:VSS) U1.56(E:VSS) U1.88(E:VSS) U1.102(E:VSS) U1.103(E:VSS) U1.115(E:VSS) U1.121(E:VSS) U1.122(E:VSS) U1.135(E:VSS) U1.138(E:VSS) U1.144(E:VSS) ; also sheet 2,3,5,7,8,9,10,11,12,13,14
VCCAD: C19.1 ; also sheet 2

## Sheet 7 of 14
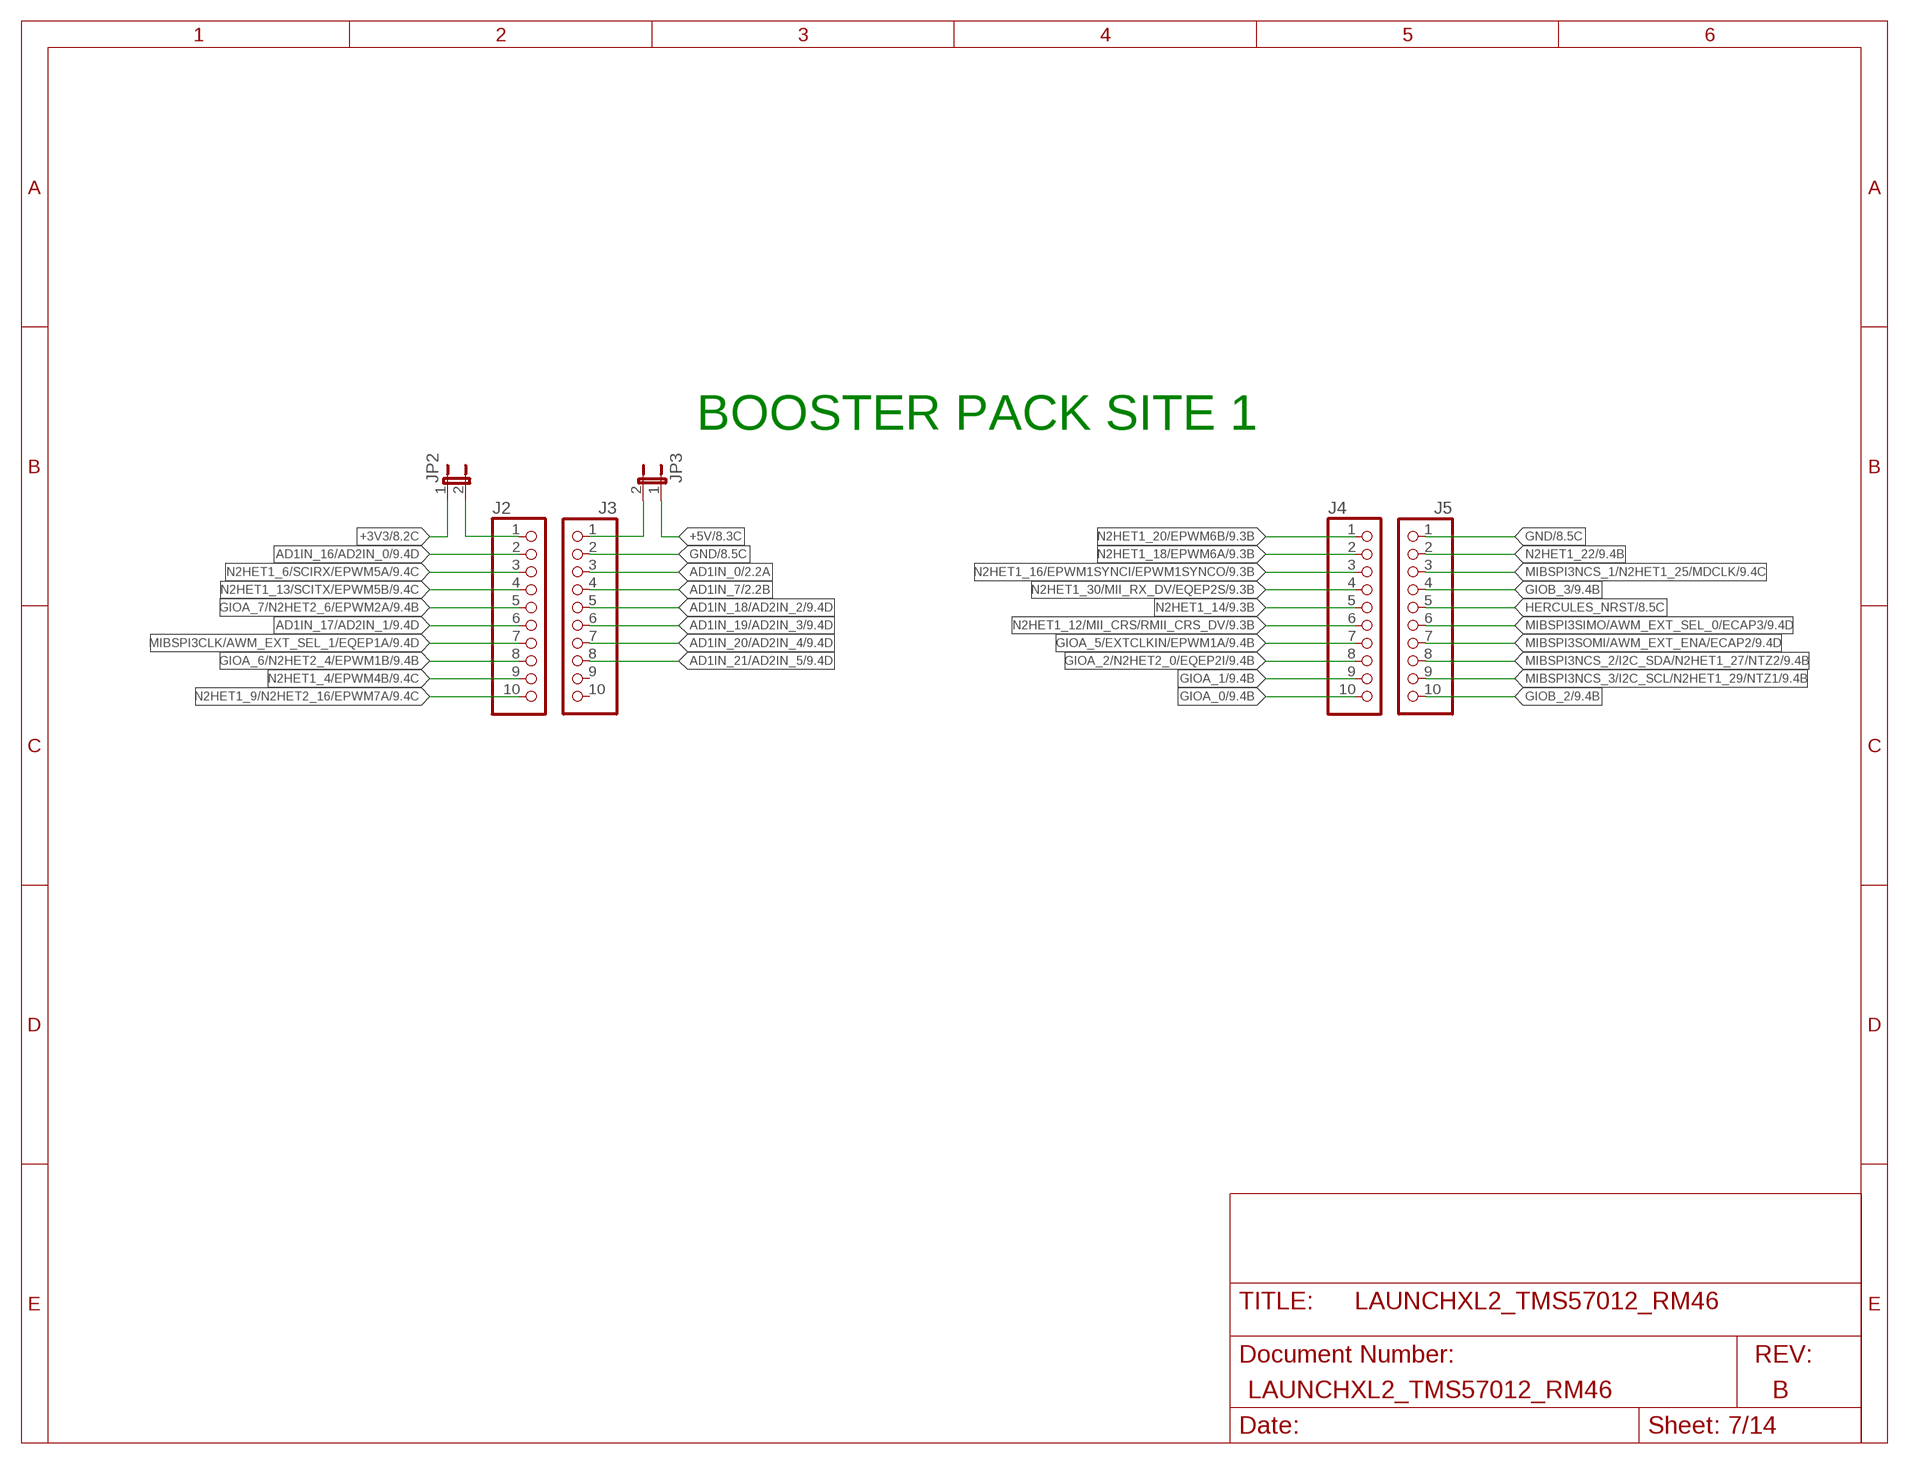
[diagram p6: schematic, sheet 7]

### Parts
J2  PINHD-1X10  [1X10]
J3  DNP* (PART OF 2X10)  PINHD-1X10  [1X10]
J4  PINHD-1X10  [1X10]
J5  DNP* (PART OF 2X10)  PINHD-1X10  [1X10]
JP2  SHUNT_ON  JP1E  [JP1]
JP3  SHUNT_ON  JP1E  [JP1]

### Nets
+3V3: JP2.1 ; also sheet 2,3,5,6,8,9,10,11,12,13
+5V: JP3.1 ; also sheet 2,8,9,11,14
AD1IN_0: J3.3 ; also sheet 2
AD1IN_7: J3.4 ; also sheet 2
AD1IN_16/AD2IN_0: J2.2 ; also sheet 2,9
AD1IN_17/AD2IN_1: J2.6 ; also sheet 2,9
AD1IN_18/AD2IN_2: J3.5 ; also sheet 2,9
AD1IN_19/AD2IN_3: J3.6 ; also sheet 2,9
AD1IN_20/AD2IN_4: J3.7 ; also sheet 2,9
AD1IN_21/AD2IN_5: J3.8 ; also sheet 2,9
GIOA_0: J4.10 ; also sheet 4,9
GIOA_1: J4.9 ; also sheet 4,9
GIOA_2/N2HET2_0/EQEP2I: J4.8 ; also sheet 4,9
GIOA_5/EXTCLKIN/EPWM1A: J4.7 ; also sheet 4,9
GIOA_6/N2HET2_4/EPWM1B: J2.8 ; also sheet 4,9
GIOA_7/N2HET2_6/EPWM2A: J2.5 ; also sheet 4,9
GIOB_2: J5.10 ; also sheet 4,9,10
GIOB_3: J5.4 ; also sheet 4,9
GND: J3.2 J5.1 ; also sheet 2,3,5,6,8,9,10,11,12,13,14
HERCULES_NRST: J5.5 ; also sheet 5,8,9,12
MIBSPI3CLK/AWM_EXT_SEL_1/EQEP1A: J2.7 ; also sheet 3,9
MIBSPI3NCS_1/N2HET1_25/MDCLK: J5.3 ; also sheet 3,9
MIBSPI3NCS_2/I2C_SDA/N2HET1_27/NTZ2: J5.8 ; also sheet 3,9
MIBSPI3NCS_3/I2C_SCL/N2HET1_29/NTZ1: J5.9 ; also sheet 3,9
MIBSPI3SIMO/AWM_EXT_SEL_0/ECAP3: J5.6 ; also sheet 3,9
MIBSPI3SOMI/AWM_EXT_ENA/ECAP2: J5.7 ; also sheet 3,9
N2HET1_4/EPWM4B: J2.9 ; also sheet 4,9
N2HET1_6/SCIRX/EPWM5A: J2.3 ; also sheet 3,9
N2HET1_9/N2HET2_16/EPWM7A: J2.10 ; also sheet 4,9
N2HET1_12/MII_CRS/RMII_CRS_DV: J4.6 ; also sheet 4,9
N2HET1_13/SCITX/EPWM5B: J2.4 ; also sheet 3,9
N2HET1_14: J4.5 ; also sheet 4,9
N2HET1_16/EPWM1SYNCI/EPWM1SYNCO: J4.3 ; also sheet 4,9
N2HET1_18/EPWM6A: J4.2 ; also sheet 4,9
N2HET1_20/EPWM6B: J4.1 ; also sheet 4,9
N2HET1_22: J5.2 ; also sheet 4,9
N2HET1_30/MII_RX_DV/EQEP2S: J4.4 ; also sheet 4,9
N$3: J2.1 JP2.2
N$4: J3.1 JP3.2
Unconnected: J3.9 J3.10

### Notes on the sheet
- BOOSTER PACK SITE 1

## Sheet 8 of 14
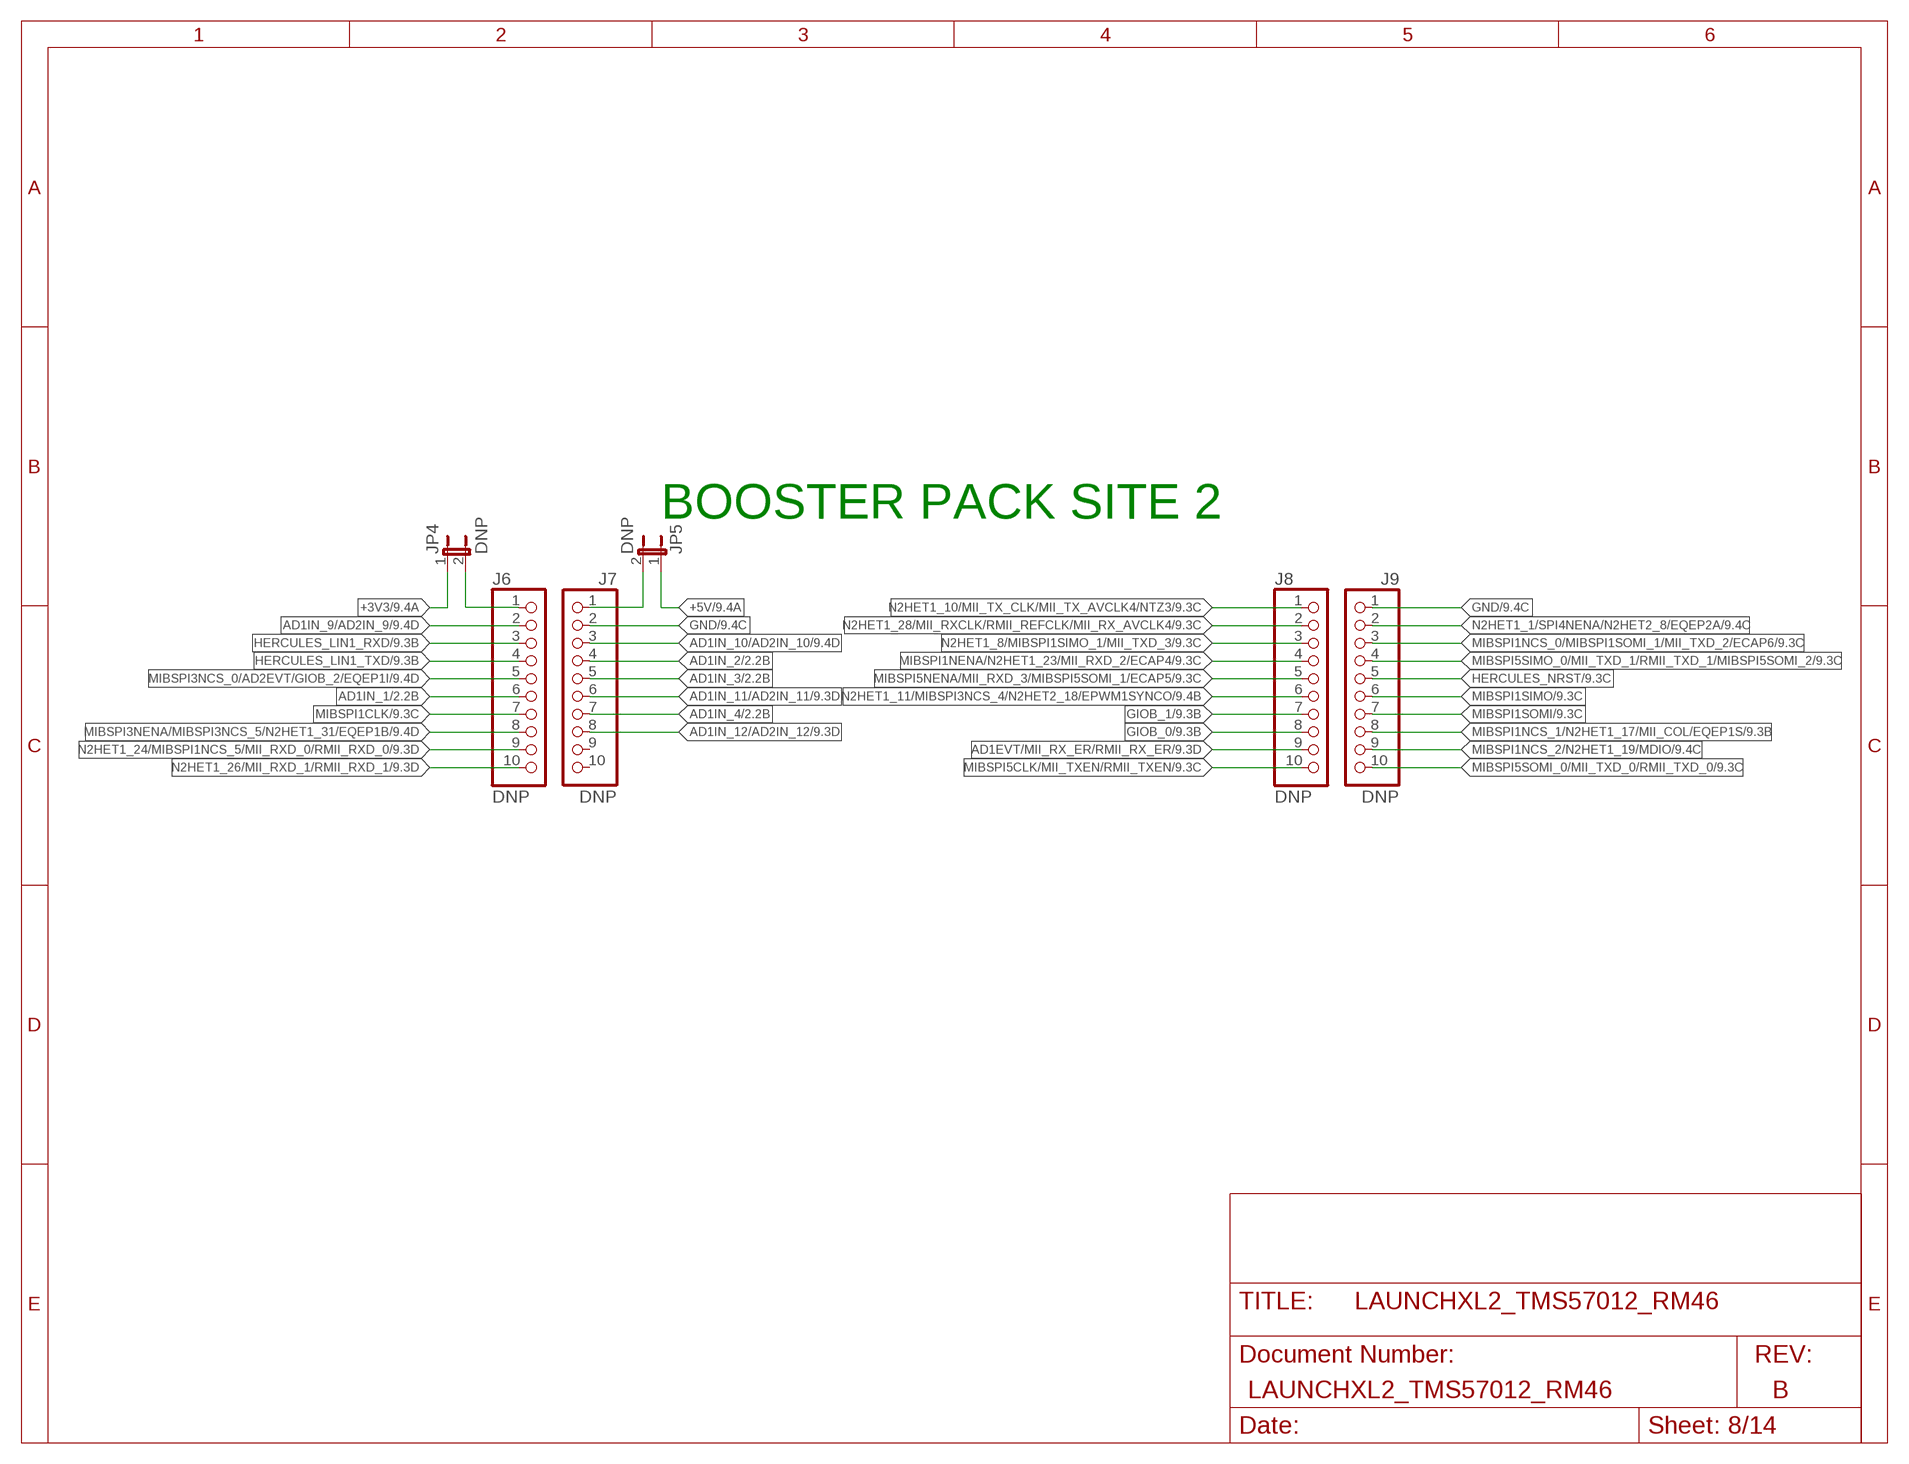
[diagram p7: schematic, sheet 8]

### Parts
J6  DNP  PINHD-1X10  [1X10]
J7  DNP  PINHD-1X10  [1X10]
J8  DNP  PINHD-1X10  [1X10]
J9  DNP  PINHD-1X10  [1X10]
JP4  DNP  JP1E  [JP1]
JP5  DNP  JP1E  [JP1]

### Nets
+3V3: JP4.1 ; also sheet 2,3,5,6,7,9,10,11,12,13
+5V: JP5.1 ; also sheet 2,7,9,11,14
AD1EVT/MII_RX_ER/RMII_RX_ER: J8.9 ; also sheet 2,9
AD1IN_1: J6.6 ; also sheet 2
AD1IN_2: J7.4 ; also sheet 2
AD1IN_3: J7.5 ; also sheet 2
AD1IN_4: J7.7 ; also sheet 2
AD1IN_9/AD2IN_9: J6.2 ; also sheet 2,9
AD1IN_10/AD2IN_10: J7.3 ; also sheet 2,9
AD1IN_11/AD2IN_11: J7.6 ; also sheet 2,9
AD1IN_12/AD2IN_12: J7.8 ; also sheet 2,9
GIOB_0: J8.8 ; also sheet 4,9
GIOB_1: J8.7 ; also sheet 4,9,10
GND: J7.2 J9.1 ; also sheet 2,3,5,6,7,9,10,11,12,13,14
HERCULES_LIN1_RXD: J6.3 ; also sheet 3,9,12
HERCULES_LIN1_TXD: J6.4 ; also sheet 3,9,12
HERCULES_NRST: J9.5 ; also sheet 5,7,9,12
MIBSPI1CLK: J6.7 ; also sheet 3,9
MIBSPI1NCS_0/MIBSPI1SOMI_1/MII_TXD_2/ECAP6: J9.3 ; also sheet 3,9
MIBSPI1NCS_1/N2HET1_17/MII_COL/EQEP1S: J9.8 ; also sheet 3,9
MIBSPI1NCS_2/N2HET1_19/MDIO: J9.9 ; also sheet 3,9
MIBSPI1NENA/N2HET1_23/MII_RXD_2/ECAP4: J8.4 ; also sheet 3,9
MIBSPI1SIMO: J9.6 ; also sheet 3,9
MIBSPI1SOMI: J9.7 ; also sheet 3,9
MIBSPI3NCS_0/AD2EVT/GIOB_2/EQEP1I: J6.5 ; also sheet 3,9,10
MIBSPI3NENA/MIBSPI3NCS_5/N2HET1_31/EQEP1B: J6.8 ; also sheet 3,9
MIBSPI5CLK/MII_TXEN/RMII_TXEN: J8.10 ; also sheet 3,9
MIBSPI5NENA/MII_RXD_3/MIBSPI5SOMI_1/ECAP5: J8.5 ; also sheet 3,9
MIBSPI5SIMO_0/MII_TXD_1/RMII_TXD_1/MIBSPI5SOMI_2: J9.4 ; also sheet 3,9
MIBSPI5SOMI_0/MII_TXD_0/RMII_TXD_0: J9.10 ; also sheet 3,9
N2HET1_1/SPI4NENA/N2HET2_8/EQEP2A: J9.2 ; also sheet 4,9
N2HET1_8/MIBSPI1SIMO_1/MII_TXD_3: J8.3 ; also sheet 4,9
N2HET1_10/MII_TX_CLK/MII_TX_AVCLK4/NTZ3: J8.1 ; also sheet 4,9
N2HET1_11/MIBSPI3NCS_4/N2HET2_18/EPWM1SYNCO: J8.6 ; also sheet 4,9
N2HET1_24/MIBSPI1NCS_5/MII_RXD_0/RMII_RXD_0: J6.9 ; also sheet 4,9
N2HET1_26/MII_RXD_1/RMII_RXD_1: J6.10 ; also sheet 4,9
N2HET1_28/MII_RXCLK/RMII_REFCLK/MII_RX_AVCLK4: J8.2 ; also sheet 4,9
N$5: J6.1 JP4.2
N$14: J7.1 JP5.2
Unconnected: J7.9 J7.10

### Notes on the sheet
- BOOSTER PACK SITE 2

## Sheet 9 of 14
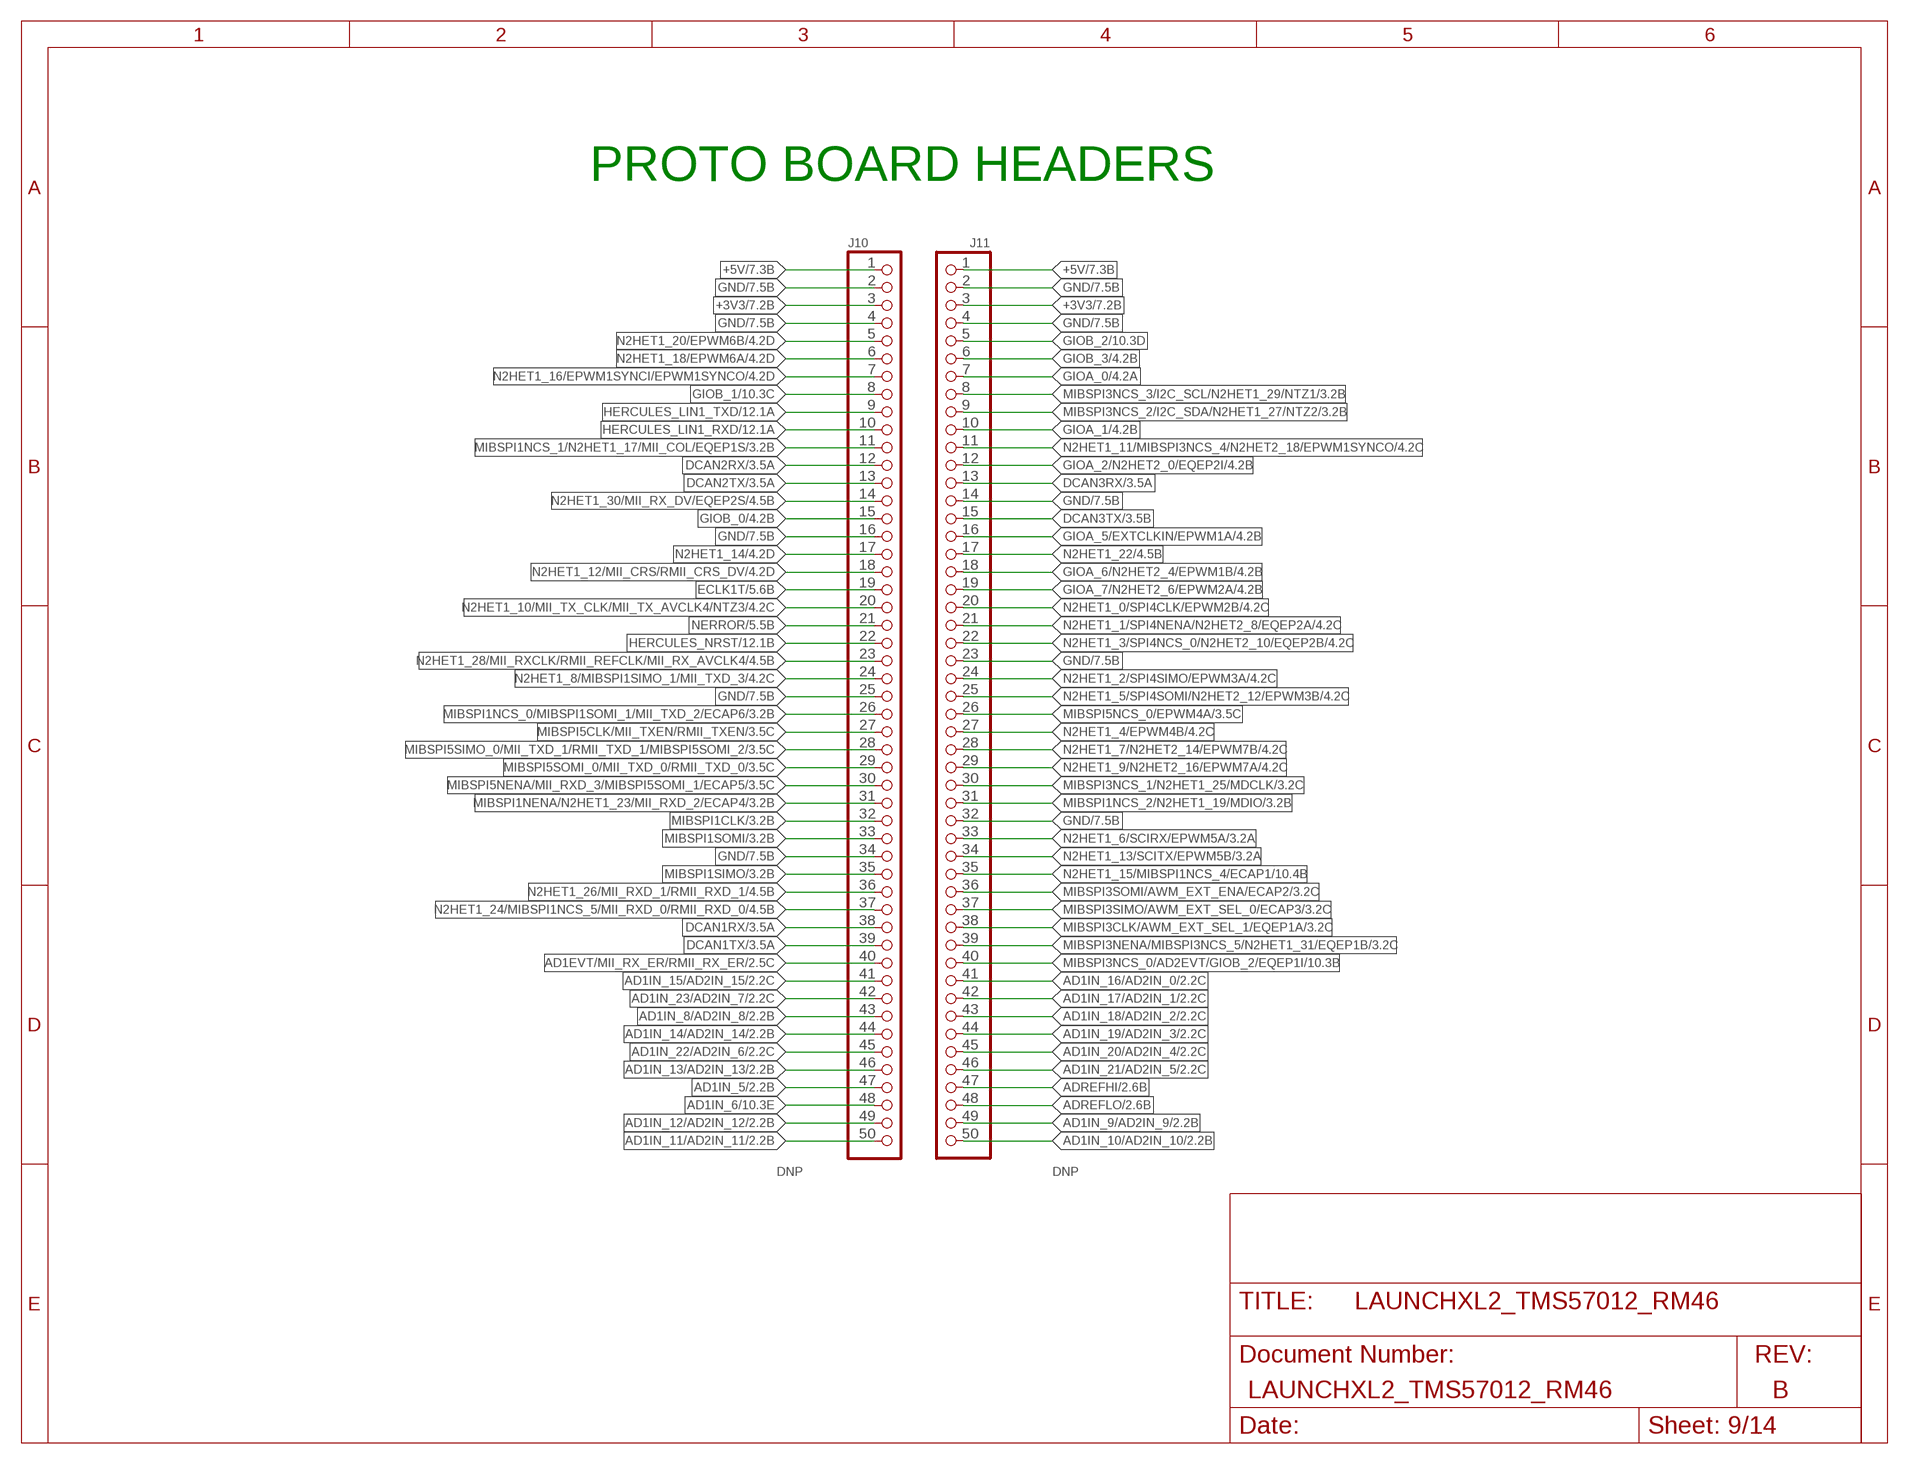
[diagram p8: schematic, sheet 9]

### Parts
J10  DNP  PINHD-1X50ALT  [1X50_ALT]
J11  DNP  PINHD-1X50  [1X50]

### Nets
+3V3: J10.3 J11.3 ; also sheet 2,3,5,6,7,8,10,11,12,13
+5V: J10.1 J11.1 ; also sheet 2,7,8,11,14
AD1EVT/MII_RX_ER/RMII_RX_ER: J10.40 ; also sheet 2,8
AD1IN_5: J10.47 ; also sheet 2
AD1IN_6: J10.48 ; also sheet 2,10
AD1IN_8/AD2IN_8: J10.43 ; also sheet 2
AD1IN_9/AD2IN_9: J11.49 ; also sheet 2,8
AD1IN_10/AD2IN_10: J11.50 ; also sheet 2,8
AD1IN_11/AD2IN_11: J10.50 ; also sheet 2,8
AD1IN_12/AD2IN_12: J10.49 ; also sheet 2,8
AD1IN_13/AD2IN_13: J10.46 ; also sheet 2
AD1IN_14/AD2IN_14: J10.44 ; also sheet 2
AD1IN_15/AD2IN_15: J10.41 ; also sheet 2
AD1IN_16/AD2IN_0: J11.41 ; also sheet 2,7
AD1IN_17/AD2IN_1: J11.42 ; also sheet 2,7
AD1IN_18/AD2IN_2: J11.43 ; also sheet 2,7
AD1IN_19/AD2IN_3: J11.44 ; also sheet 2,7
AD1IN_20/AD2IN_4: J11.45 ; also sheet 2,7
AD1IN_21/AD2IN_5: J11.46 ; also sheet 2,7
AD1IN_22/AD2IN_6: J10.45 ; also sheet 2
AD1IN_23/AD2IN_7: J10.42 ; also sheet 2
ADREFHI: J11.47 ; also sheet 2
ADREFLO: J11.48 ; also sheet 2
DCAN1RX: J10.38 ; also sheet 3
DCAN1TX: J10.39 ; also sheet 3
DCAN2RX: J10.12 ; also sheet 3
DCAN2TX: J10.13 ; also sheet 3
DCAN3RX: J11.13 ; also sheet 3
DCAN3TX: J11.15 ; also sheet 3
ECLK1T: J10.19 ; also sheet 5
GIOA_0: J11.7 ; also sheet 4,7
GIOA_1: J11.10 ; also sheet 4,7
GIOA_2/N2HET2_0/EQEP2I: J11.12 ; also sheet 4,7
GIOA_5/EXTCLKIN/EPWM1A: J11.16 ; also sheet 4,7
GIOA_6/N2HET2_4/EPWM1B: J11.18 ; also sheet 4,7
GIOA_7/N2HET2_6/EPWM2A: J11.19 ; also sheet 4,7
GIOB_0: J10.15 ; also sheet 4,8
GIOB_1: J10.8 ; also sheet 4,8,10
GIOB_2: J11.5 ; also sheet 4,7,10
GIOB_3: J11.6 ; also sheet 4,7
GND: J10.2 J10.4 J10.16 J10.25 J10.34 J11.2 J11.4 J11.14 J11.23 J11.32 ; also sheet 2,3,5,6,7,8,10,11,12,13,14
HERCULES_LIN1_RXD: J10.10 ; also sheet 3,8,12
HERCULES_LIN1_TXD: J10.9 ; also sheet 3,8,12
HERCULES_NRST: J10.22 ; also sheet 5,7,8,12
MIBSPI1CLK: J10.32 ; also sheet 3,8
MIBSPI1NCS_0/MIBSPI1SOMI_1/MII_TXD_2/ECAP6: J10.26 ; also sheet 3,8
MIBSPI1NCS_1/N2HET1_17/MII_COL/EQEP1S: J10.11 ; also sheet 3,8
MIBSPI1NCS_2/N2HET1_19/MDIO: J11.31 ; also sheet 3,8
MIBSPI1NENA/N2HET1_23/MII_RXD_2/ECAP4: J10.31 ; also sheet 3,8
MIBSPI1SIMO: J10.35 ; also sheet 3,8
MIBSPI1SOMI: J10.33 ; also sheet 3,8
MIBSPI3CLK/AWM_EXT_SEL_1/EQEP1A: J11.38 ; also sheet 3,7
MIBSPI3NCS_0/AD2EVT/GIOB_2/EQEP1I: J11.40 ; also sheet 3,8,10
MIBSPI3NCS_1/N2HET1_25/MDCLK: J11.30 ; also sheet 3,7
MIBSPI3NCS_2/I2C_SDA/N2HET1_27/NTZ2: J11.9 ; also sheet 3,7
MIBSPI3NCS_3/I2C_SCL/N2HET1_29/NTZ1: J11.8 ; also sheet 3,7
MIBSPI3NENA/MIBSPI3NCS_5/N2HET1_31/EQEP1B: J11.39 ; also sheet 3,8
MIBSPI3SIMO/AWM_EXT_SEL_0/ECAP3: J11.37 ; also sheet 3,7
MIBSPI3SOMI/AWM_EXT_ENA/ECAP2: J11.36 ; also sheet 3,7
MIBSPI5CLK/MII_TXEN/RMII_TXEN: J10.27 ; also sheet 3,8
MIBSPI5NCS_0/EPWM4A: J11.26 ; also sheet 3
MIBSPI5NENA/MII_RXD_3/MIBSPI5SOMI_1/ECAP5: J10.30 ; also sheet 3,8
MIBSPI5SIMO_0/MII_TXD_1/RMII_TXD_1/MIBSPI5SOMI_2: J10.28 ; also sheet 3,8
MIBSPI5SOMI_0/MII_TXD_0/RMII_TXD_0: J10.29 ; also sheet 3,8
N2HET1_0/SPI4CLK/EPWM2B: J11.20 ; also sheet 4
N2HET1_1/SPI4NENA/N2HET2_8/EQEP2A: J11.21 ; also sheet 4,8
N2HET1_2/SPI4SIMO/EPWM3A: J11.24 ; also sheet 4
N2HET1_3/SPI4NCS_0/N2HET2_10/EQEP2B: J11.22 ; also sheet 4
N2HET1_4/EPWM4B: J11.27 ; also sheet 4,7
N2HET1_5/SPI4SOMI/N2HET2_12/EPWM3B: J11.25 ; also sheet 4
N2HET1_6/SCIRX/EPWM5A: J11.33 ; also sheet 3,7
N2HET1_7/N2HET2_14/EPWM7B: J11.28 ; also sheet 4
N2HET1_8/MIBSPI1SIMO_1/MII_TXD_3: J10.24 ; also sheet 4,8
N2HET1_9/N2HET2_16/EPWM7A: J11.29 ; also sheet 4,7
N2HET1_10/MII_TX_CLK/MII_TX_AVCLK4/NTZ3: J10.20 ; also sheet 4,8
N2HET1_11/MIBSPI3NCS_4/N2HET2_18/EPWM1SYNCO: J11.11 ; also sheet 4,8
N2HET1_12/MII_CRS/RMII_CRS_DV: J10.18 ; also sheet 4,7
N2HET1_13/SCITX/EPWM5B: J11.34 ; also sheet 3,7
N2HET1_14: J10.17 ; also sheet 4,7
N2HET1_15/MIBSPI1NCS_4/ECAP1: J11.35 ; also sheet 4,10
N2HET1_16/EPWM1SYNCI/EPWM1SYNCO: J10.7 ; also sheet 4,7
N2HET1_18/EPWM6A: J10.6 ; also sheet 4,7
N2HET1_20/EPWM6B: J10.5 ; also sheet 4,7
N2HET1_22: J11.17 ; also sheet 4,7
N2HET1_24/MIBSPI1NCS_5/MII_RXD_0/RMII_RXD_0: J10.37 ; also sheet 4,8
N2HET1_26/MII_RXD_1/RMII_RXD_1: J10.36 ; also sheet 4,8
N2HET1_28/MII_RXCLK/RMII_REFCLK/MII_RX_AVCLK4: J10.23 ; also sheet 4,8
N2HET1_30/MII_RX_DV/EQEP2S: J10.14 ; also sheet 4,7
NERROR: J10.21 ; also sheet 5

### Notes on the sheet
- PROTO BOARD HEADERS

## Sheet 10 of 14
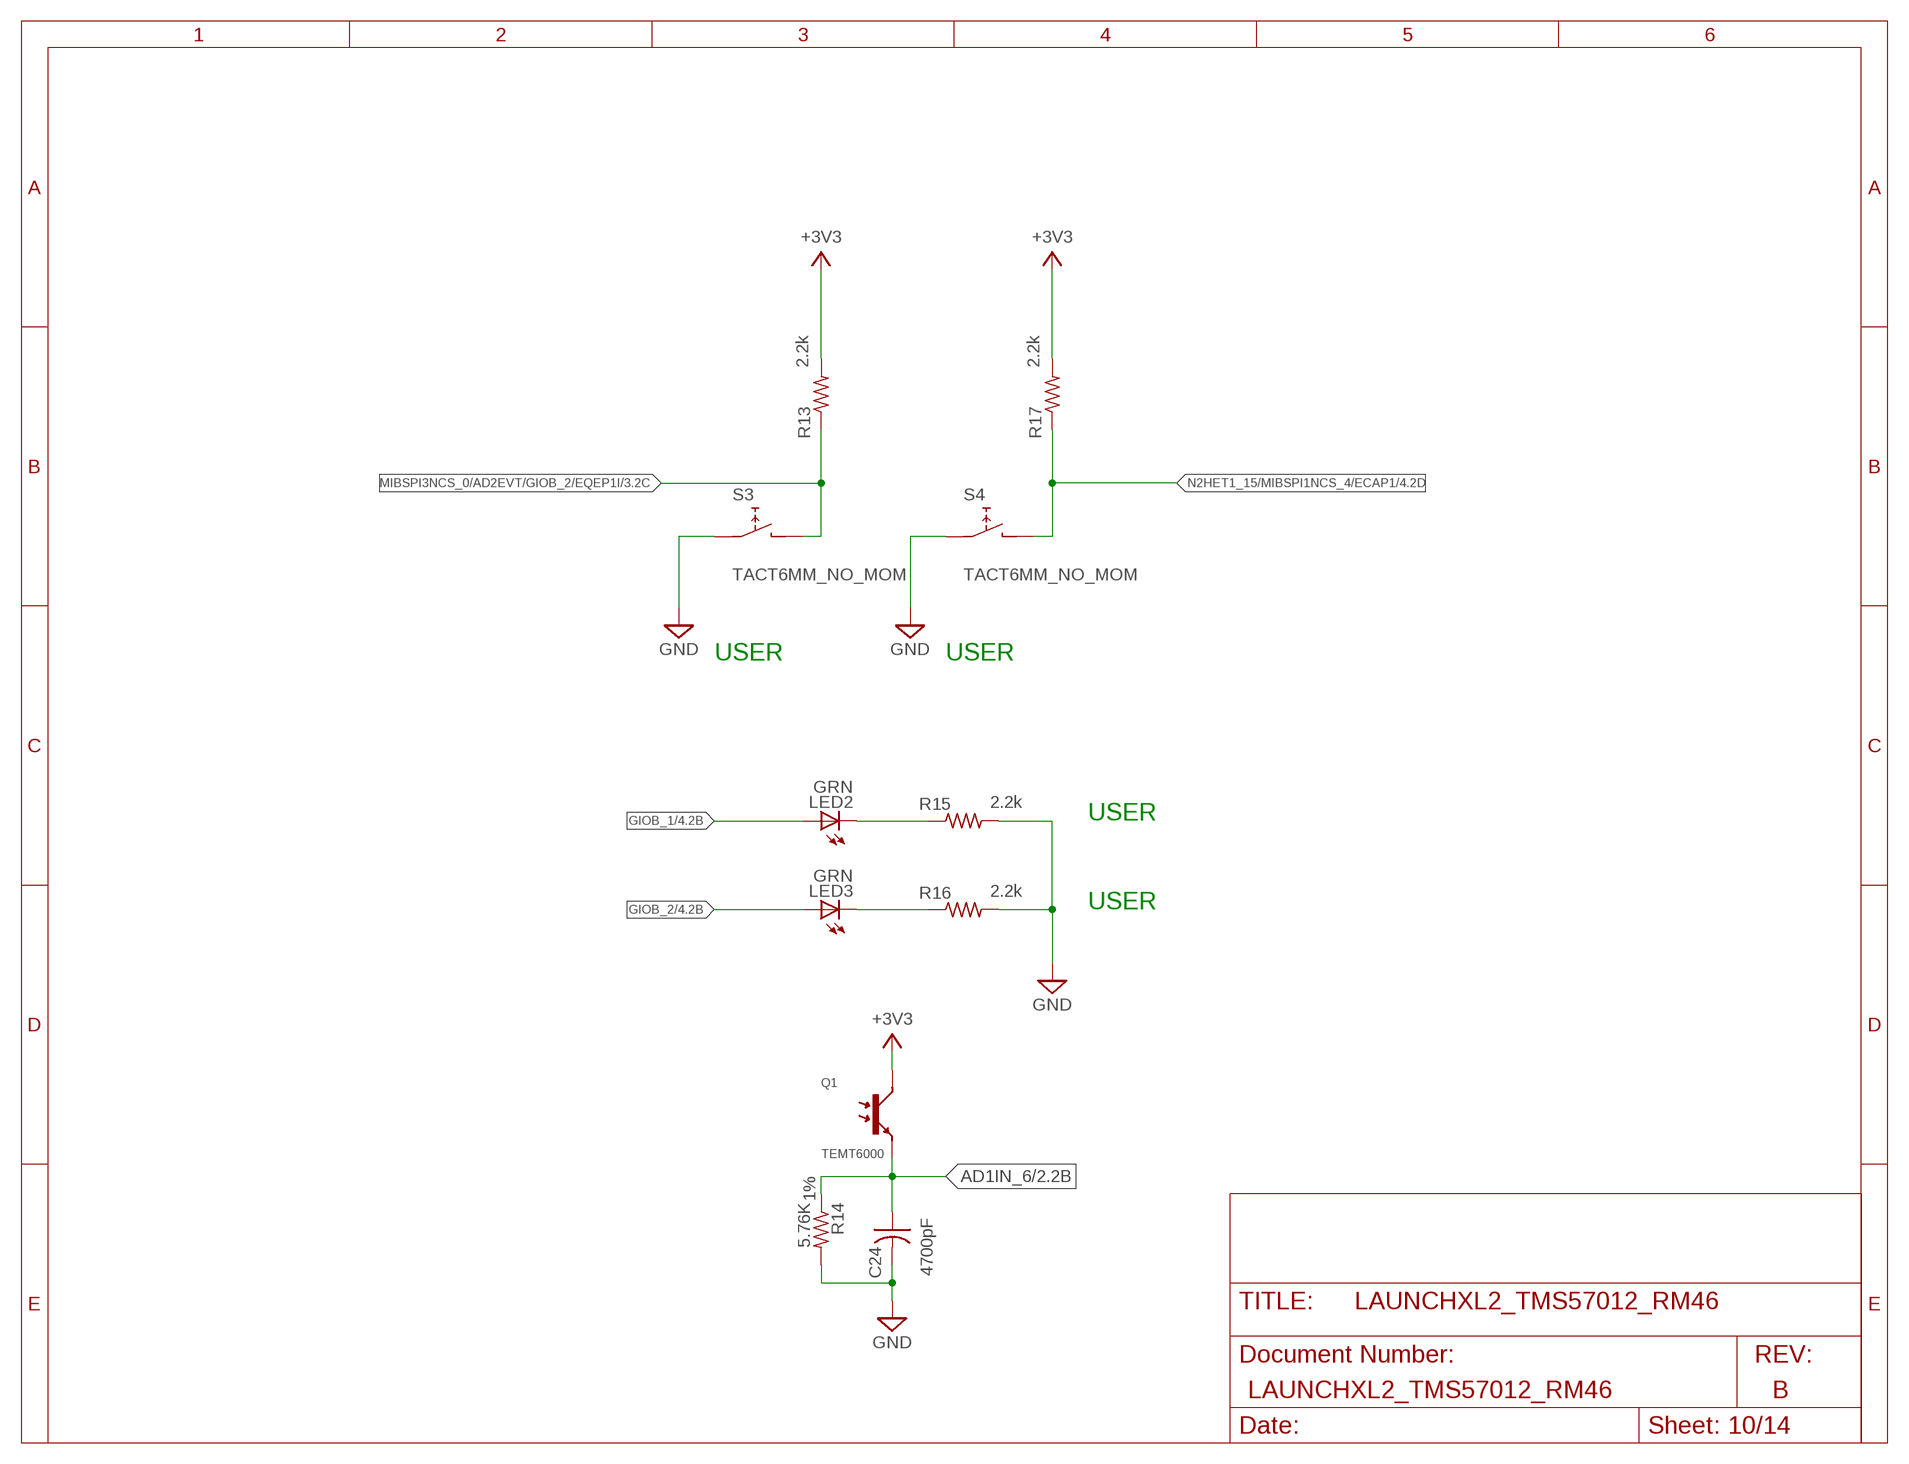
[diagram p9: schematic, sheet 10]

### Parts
C24  4700pF  C-USC0402K  [C0402K]
LED2  GRN  LEDCHIPLED_0603  [CHIPLED_0603]
LED3  GRN  LEDCHIPLED_0603  [CHIPLED_0603]
Q1  TEMT6000  [TEMT6000]
R13  2.2k  R-US_R0402  [R0402]
R14  5.76K  R-US_R0402  [R0402]
R15  2.2k  R-US_R0402  [R0402]
R16  2.2k  R-US_R0402  [R0402]
R17  2.2k  R-US_R0402  [R0402]
S3  TACT6MM_NO_MOM  [CK_PTS645_SMD]
S4  TACT6MM_NO_MOM  [CK_PTS645_SMD]

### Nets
+3V3: Q1.3(C) R13.2 R17.2 ; also sheet 2,3,5,6,7,8,9,11,12,13
AD1IN_6: C24.1 Q1.1(E) R14.1 ; also sheet 2,9
GIOB_1: LED2.A ; also sheet 4,8,9
GIOB_2: LED3.A ; also sheet 4,7,9
GND: C24.2 R14.2 R15.2 R16.2 S3.1 S3.2 S4.1 S4.2 ; also sheet 2,3,5,6,7,8,9,11,12,13,14
MIBSPI3NCS_0/AD2EVT/GIOB_2/EQEP1I: R13.1 S3.3 S3.4 ; also sheet 3,8,9
N2HET1_15/MIBSPI1NCS_4/ECAP1: R17.1 S4.3 S4.4 ; also sheet 4,9
N$35: LED3.C R16.1
N$36: LED2.C R15.1
Unconnected: Q1.2(NC)

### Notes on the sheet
- USER | USER
- USER
- USER

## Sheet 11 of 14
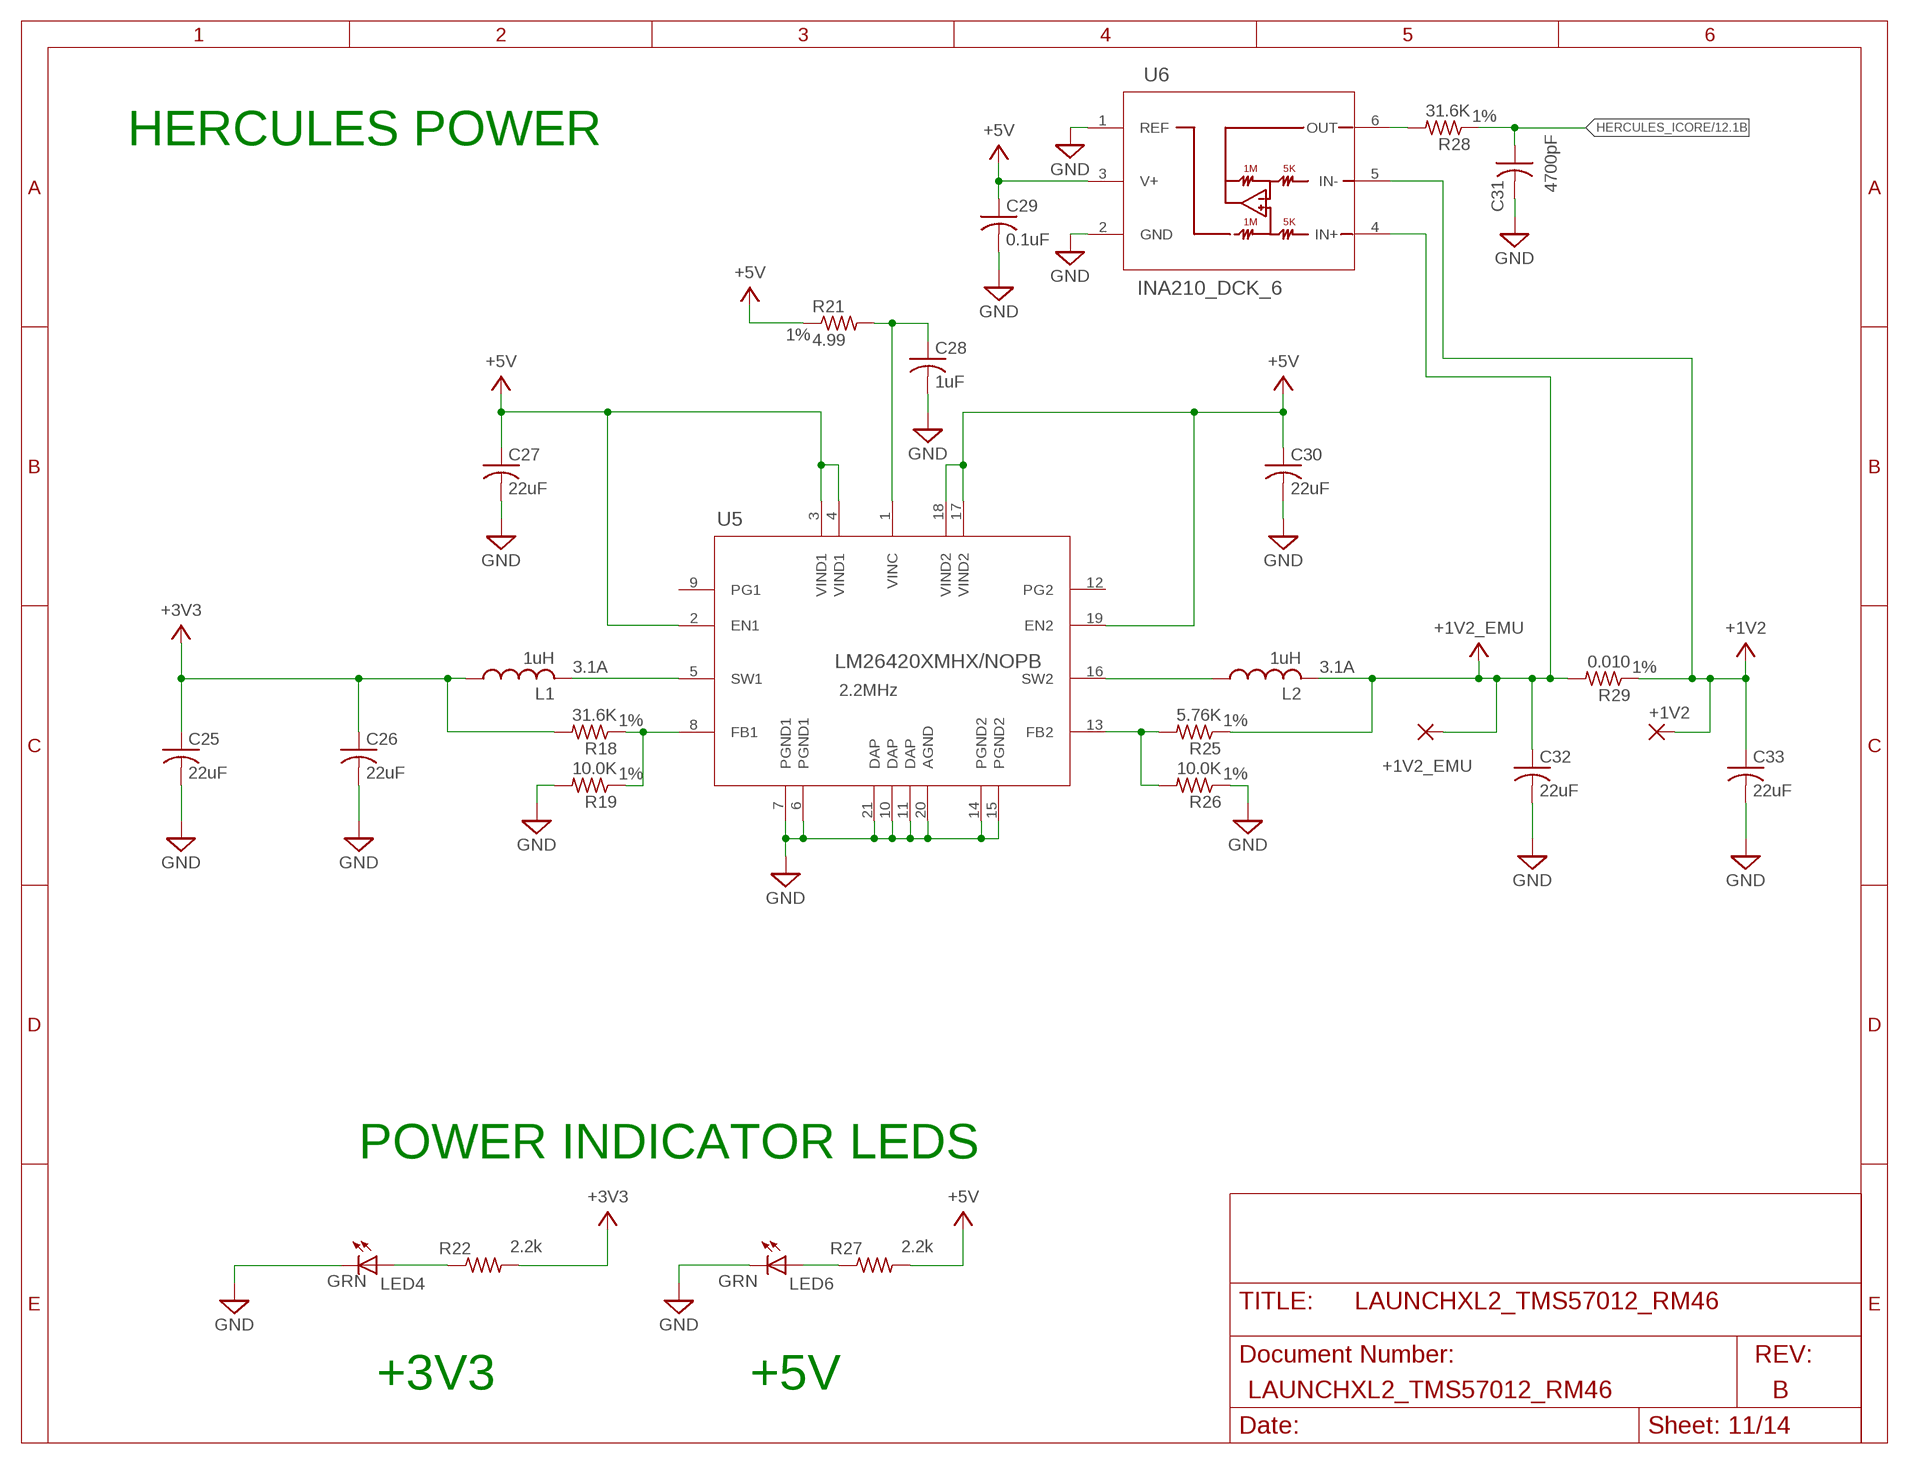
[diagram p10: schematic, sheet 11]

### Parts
+1V2  DNP  WIREPAD1,6/0,9  [1,6/0,9]
+1V2_EMU  DNP  WIREPAD1,6/0,9  [1,6/0,9]
C25  22uF  C-USC0805K  [C0805K]
C26  22uF  C-USC0805K  [C0805K]
C27  22uF  C-USC0805K  [C0805K]
C28  1uF  C-USC0402K  [C0402K]
C29  0.1uF  C-USC0402K  [C0402K]
C30  22uF  C-USC0805K  [C0805K]
C31  4700pF  C-USC0402K  [C0402K]
C32  22uF  C-USC0805K  [C0805K]
C33  22uF  C-USC0805K  [C0805K]
L1  1uH  L-USL2520P  [L2520P]
L2  1uH  L-USL2520P  [L2520P]
LED4  GRN  LEDCHIPLED_0603  [CHIPLED_0603]
LED6  GRN  LEDCHIPLED_0603  [CHIPLED_0603]
R18  31.6K  R-US_R0402  [R0402]
R19  10.0K  R-US_R0402  [R0402]
R21  4.99  R-US_R0402  [R0402]
R22  2.2k  R-US_R0402  [R0402]
R25  5.76K  R-US_R0402  [R0402]
R26  10.0K  R-US_R0402  [R0402]
R27  2.2k  R-US_R0402  [R0402]
R28  31.6K  R-US_R0402  [R0402]
R29  0.010  R-US_R1206W  [R1206W]
U5  LM26420XMHX/NOPB  LM26420_PWP_20  [MXA20A]
U6  INA210_DCK_6  [DCK6]

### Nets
+1V2: +1V2.1(P) C33.1 R29.1 U6.5(IN-) ; also sheet 5,6,12
+1V2_EMU: +1V2_EMU.1(P) C32.1 L2.2 R25.1 R29.2 U6.4(IN+)
+3V3: C25.1 C26.1 L1.1 R18.2 R22.2 ; also sheet 2,3,5,6,7,8,9,10,12,13
+5V: C27.1 C29.1 C30.1 R21.1 R27.2 U5.2(EN1) U5.3(VIND1) U5.4(VIND1) U5.17(VIND2) U5.18(VIND2) U5.19(EN2) U6.3(V+) ; also sheet 2,7,8,9,14
GND: C25.2 C26.2 C27.2 C28.2 C29.2 C30.2 C31.2 C32.2 C33.2 LED4.C LED6.C R19.2 R26.1 U5.6(PGND1) U5.7(PGND1) U5.10(DAP) U5.11(DAP) U5.14(PGND2) U5.15(PGND2) U5.20(AGND) U5.21(DAP) U6.1(REF) U6.2(GND) ; also sheet 2,3,5,6,7,8,9,10,12,13,14
HERCULES_ICORE: C31.1 R28.1 ; also sheet 12
N$9: L1.2 U5.5(SW1)
N$11: R18.1 R19.1 U5.8(FB1)
N$12: L2.1 U5.16(SW2)
N$13: C28.1 R21.2 U5.1(VINC)
N$16: LED6.A R27.1
N$17: R25.2 R26.2 U5.13(FB2)
N$21: LED4.A R22.1
N$41: R28.2 U6.6(OUT)
Unconnected: U5.9(PG1) U5.12(PG2)

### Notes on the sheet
- HERCULES POWER
- POWER INDICATOR LEDS
- +3V3 | +5V

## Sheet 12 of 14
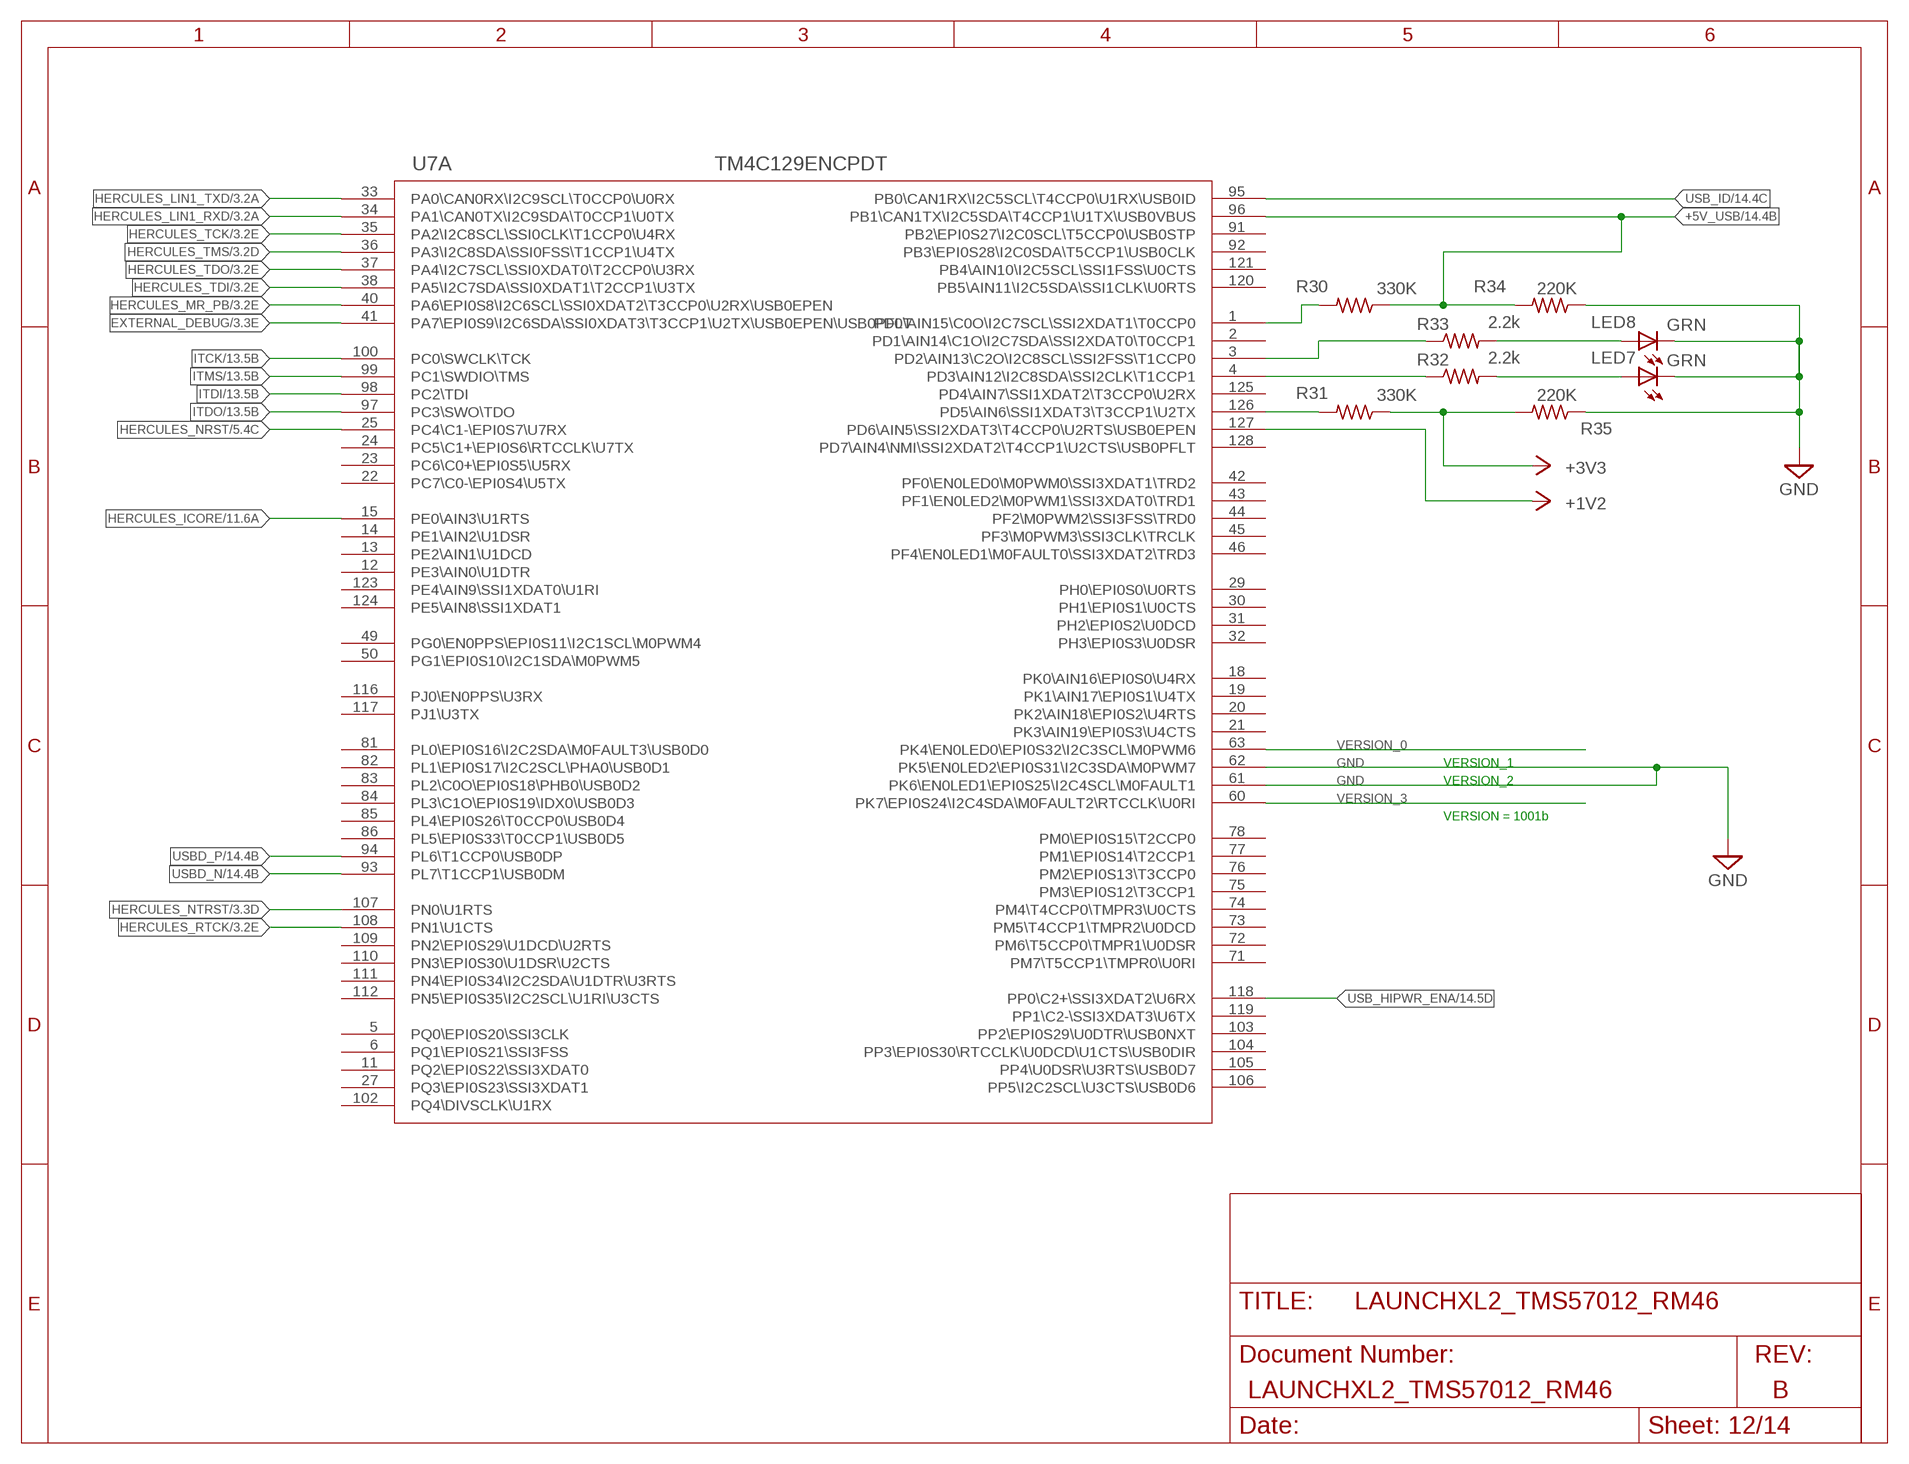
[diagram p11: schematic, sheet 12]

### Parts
LED7  GRN  LEDCHIPLED_0603  [CHIPLED_0603]
LED8  GRN  LEDCHIPLED_0603  [CHIPLED_0603]
R30  330K  R-US_R0402  [R0402]
R31  330K  R-US_R0402  [R0402]
R32  2.2k  R-US_R0402  [R0402]
R33  2.2k  R-US_R0402  [R0402]
R34  220K  R-US_R0402  [R0402]
R35  220K  R-US_R0402  [R0402]
U7  TM4C129ENCPDT  [PDT128]

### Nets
+1V2: U7.127(A:PD6\AIN5\SSI2XDAT3\T4CCP0\U2RTS\USB0EPEN) ; also sheet 5,6,11
+3V3: R31.1 R35.2 ; also sheet 2,3,5,6,7,8,9,10,11,13
+5V_USB: R30.1 R34.2 U7.96(A:PB1\CAN1TX\I2C5SDA\T4CCP1\U1TX\USB0VBUS) ; also sheet 14
EXTERNAL_DEBUG: U7.41(A:PA7\EPI0S9\I2C6SDA\SSI0XDAT3\T3CCP1\U2TX\USB0EPEN\USB0PFLT) ; also sheet 3
GND: LED7.C LED8.C R34.1 R35.1 U7.61(A:PK6\EN0LED1\EPI0S25\I2C4SCL\M0FAULT1) U7.62(A:PK5\EN0LED2\EPI0S31\I2C3SDA\M0PWM7) ; also sheet 2,3,5,6,7,8,9,10,11,13,14
HERCULES_ICORE: U7.15(A:PE0\AIN3\U1RTS) ; also sheet 11
HERCULES_LIN1_RXD: U7.34(A:PA1\CAN0TX\I2C9SDA\T0CCP1\U0TX) ; also sheet 3,8,9
HERCULES_LIN1_TXD: U7.33(A:PA0\CAN0RX\I2C9SCL\T0CCP0\U0RX) ; also sheet 3,8,9
HERCULES_MR_PB: U7.40(A:PA6\EPI0S8\I2C6SCL\SSI0XDAT2\T3CCP0\U2RX\USB0EPEN) ; also sheet 3,5
HERCULES_NRST: U7.25(A:PC4\C1-\EPI0S7\U7RX) ; also sheet 5,7,8,9
HERCULES_NTRST: U7.107(A:PN0\U1RTS) ; also sheet 3
HERCULES_RTCK: U7.108(A:PN1\U1CTS) ; also sheet 3
HERCULES_TCK: U7.35(A:PA2\I2C8SCL\SSI0CLK\T1CCP0\U4RX) ; also sheet 3
HERCULES_TDI: U7.38(A:PA5\I2C7SDA\SSI0XDAT1\T2CCP1\U3TX) ; also sheet 3
HERCULES_TDO: U7.37(A:PA4\I2C7SCL\SSI0XDAT0\T2CCP0\U3RX) ; also sheet 3
HERCULES_TMS: U7.36(A:PA3\I2C8SDA\SSI0FSS\T1CCP1\U4TX) ; also sheet 3
ITCK: U7.100(A:PC0\SWCLK\TCK) ; also sheet 13
ITDI: U7.98(A:PC2\TDI) ; also sheet 13
ITDO: U7.97(A:PC3\SWO\TDO) ; also sheet 13
ITMS: U7.99(A:PC1\SWDIO\TMS) ; also sheet 13
N$1: R32.1 U7.4(A:PD3\AIN12\I2C8SDA\SSI2CLK\T1CCP1)
N$2: LED7.A R32.2
N$6: R33.1 U7.3(A:PD2\AIN13\C2O\I2C8SCL\SSI2FSS\T1CCP0)
N$43: R30.2 U7.1(A:PD0\AIN15\C0O\I2C7SCL\SSI2XDAT1\T0CCP0)
N$58: LED8.A R33.2
N$59: R31.2 U7.126(A:PD5\AIN6\SSI1XDAT3\T3CCP1\U2TX)
USB_HIPWR_ENA: U7.118(A:PP0\C2+\SSI3XDAT2\U6RX) ; also sheet 14
USB_ID: U7.95(A:PB0\CAN1RX\I2C5SCL\T4CCP0\U1RX\USB0ID) ; also sheet 14
USBD_N [USBD]: U7.93(A:PL7\T1CCP1\USB0DM) ; also sheet 14
USBD_P [USBD]: U7.94(A:PL6\T1CCP0\USB0DP) ; also sheet 14
VERSION_0: U7.63(A:PK4\EN0LED0\EPI0S32\I2C3SCL\M0PWM6)
VERSION_3: U7.60(A:PK7\EPI0S24\I2C4SDA\M0FAULT2\RTCCLK\U0RI)
Unconnected: U7.2(A:PD1\AIN14\C1O\I2C7SDA\SSI2XDAT0\T0CCP1) U7.5(A:PQ0\EPI0S20\SSI3CLK) U7.6(A:PQ1\EPI0S21\SSI3FSS) U7.11(A:PQ2\EPI0S22\SSI3XDAT0) U7.12(A:PE3\AIN0\U1DTR) U7.13(A:PE2\AIN1\U1DCD) U7.14(A:PE1\AIN2\U1DSR) U7.18(A:PK0\AIN16\EPI0S0\U4RX) U7.19(A:PK1\AIN17\EPI0S1\U4TX) U7.20(A:PK2\AIN18\EPI0S2\U4RTS) U7.21(A:PK3\AIN19\EPI0S3\U4CTS) U7.22(A:PC7\C0-\EPI0S4\U5TX) U7.23(A:PC6\C0+\EPI0S5\U5RX) U7.24(A:PC5\C1+\EPI0S6\RTCCLK\U7TX) U7.27(A:PQ3\EPI0S23\SSI3XDAT1) U7.29(A:PH0\EPI0S0\U0RTS) U7.30(A:PH1\EPI0S1\U0CTS) U7.31(A:PH2\EPI0S2\U0DCD) U7.32(A:PH3\EPI0S3\U0DSR) U7.42(A:PF0\EN0LED0\M0PWM0\SSI3XDAT1\TRD2) U7.43(A:PF1\EN0LED2\M0PWM1\SSI3XDAT0\TRD1) U7.44(A:PF2\M0PWM2\SSI3FSS\TRD0) U7.45(A:PF3\M0PWM3\SSI3CLK\TRCLK) U7.46(A:PF4\EN0LED1\M0FAULT0\SSI3XDAT2\TRD3) U7.49(A:PG0\EN0PPS\EPI0S11\I2C1SCL\M0PWM4) U7.50(A:PG1\EPI0S10\I2C1SDA\M0PWM5) U7.71(A:PM7\T5CCP1\TMPR0\U0RI) U7.72(A:PM6\T5CCP0\TMPR1\U0DSR) U7.73(A:PM5\T4CCP1\TMPR2\U0DCD) U7.74(A:PM4\T4CCP0\TMPR3\U0CTS) U7.75(A:PM3\EPI0S12\T3CCP1) U7.76(A:PM2\EPI0S13\T3CCP0) U7.77(A:PM1\EPI0S14\T2CCP1) U7.78(A:PM0\EPI0S15\T2CCP0) U7.81(A:PL0\EPI0S16\I2C2SDA\M0FAULT3\USB0D0) U7.82(A:PL1\EPI0S17\I2C2SCL\PHA0\USB0D1) U7.83(A:PL2\C0O\EPI0S18\PHB0\USB0D2) U7.84(A:PL3\C1O\EPI0S19\IDX0\USB0D3) U7.85(A:PL4\EPI0S26\T0CCP0\USB0D4) U7.86(A:PL5\EPI0S33\T0CCP1\USB0D5) U7.91(A:PB2\EPI0S27\I2C0SCL\T5CCP0\USB0STP) U7.92(A:PB3\EPI0S28\I2C0SDA\T5CCP1\USB0CLK) U7.102(A:PQ4\DIVSCLK\U1RX) U7.103(A:PP2\EPI0S29\U0DTR\USB0NXT) U7.104(A:PP3\EPI0S30\RTCCLK\U0DCD\U1CTS\USB0DIR) U7.105(A:PP4\U0DSR\U3RTS\USB0D7) U7.106(A:PP5\I2C2SCL\U3CTS\USB0D6) U7.109(A:PN2\EPI0S29\U1DCD\U2RTS) U7.110(A:PN3\EPI0S30\U1DSR\U2CTS) U7.111(A:PN4\EPI0S34\I2C2SDA\U1DTR\U3RTS) U7.112(A:PN5\EPI0S35\I2C2SCL\U1RI\U3CTS) U7.116(A:PJ0\EN0PPS\U3RX) U7.117(A:PJ1\U3TX) U7.119(A:PP1\C2-\SSI3XDAT3\U6TX) U7.120(A:PB5\AIN11\I2C5SDA\SSI1CLK\U0RTS) U7.121(A:PB4\AIN10\I2C5SCL\SSI1FSS\U0CTS) U7.123(A:PE4\AIN9\SSI1XDAT0\U1RI) U7.124(A:PE5\AIN8\SSI1XDAT1) U7.125(A:PD4\AIN7\SSI1XDAT2\T3CCP0\U2RX) U7.128(A:PD7\AIN4\NMI\SSI2XDAT2\T4CCP1\U2CTS\USB0PFLT)

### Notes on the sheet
- VERSION_1
- VERSION_2
- VERSION = 1001b

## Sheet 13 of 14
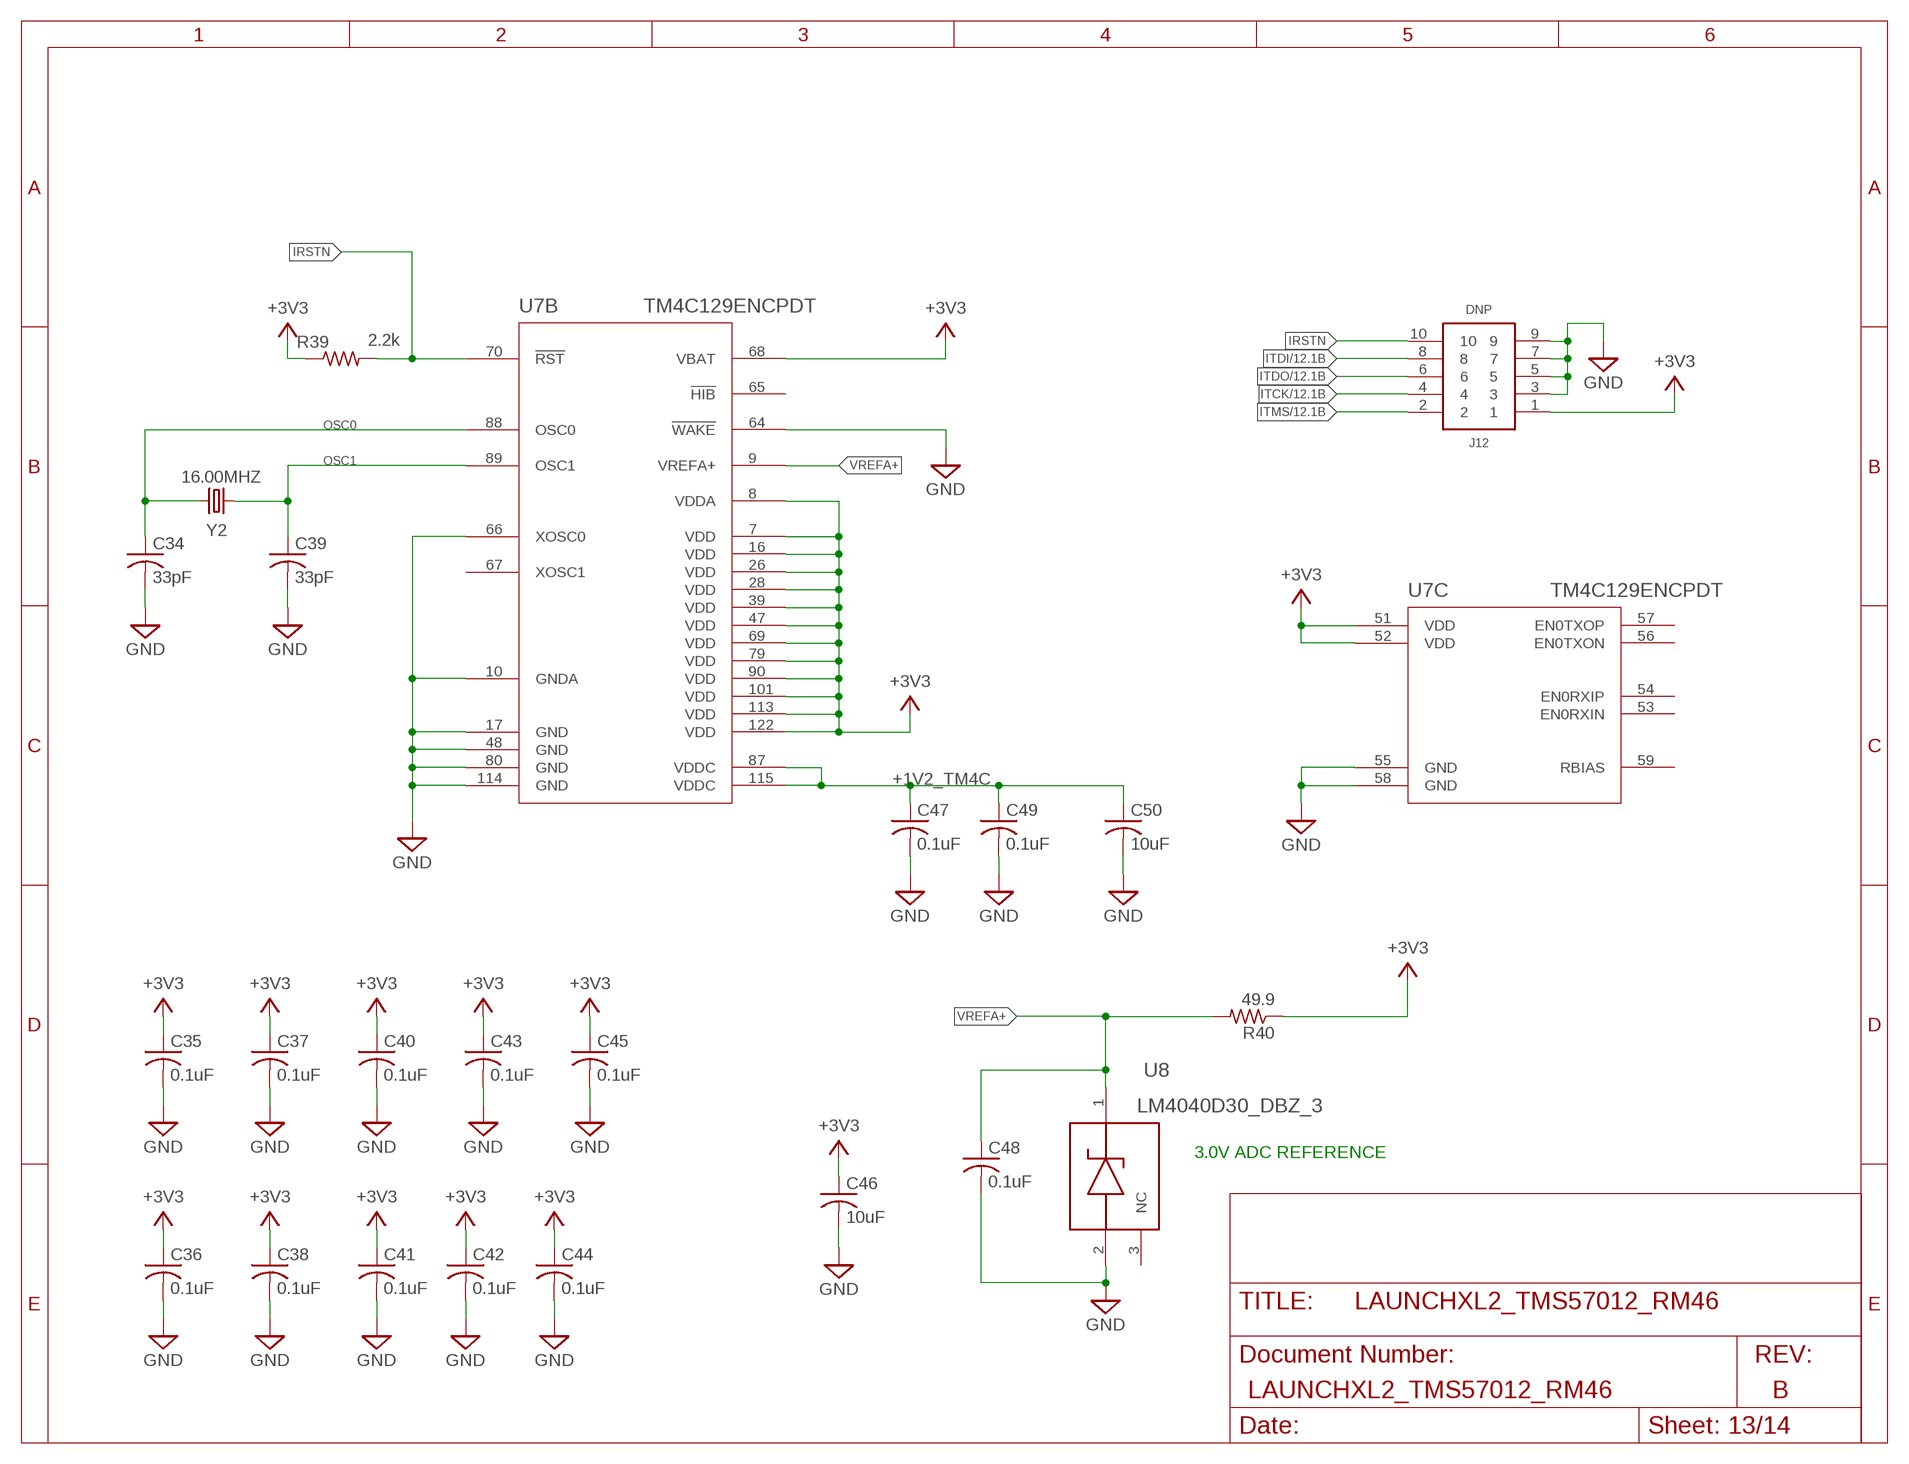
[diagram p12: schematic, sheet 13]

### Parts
C34  33pF  C-USC0402K  [C0402K]
C35  0.1uF  C-USC0402K  [C0402K]
C36  0.1uF  C-USC0402K  [C0402K]
C37  0.1uF  C-USC0402K  [C0402K]
C38  0.1uF  C-USC0402K  [C0402K]
C39  33pF  C-USC0402K  [C0402K]
C40  0.1uF  C-USC0402K  [C0402K]
C41  0.1uF  C-USC0402K  [C0402K]
C42  0.1uF  C-USC0402K  [C0402K]
C43  0.1uF  C-USC0402K  [C0402K]
C44  0.1uF  C-USC0402K  [C0402K]
C45  0.1uF  C-USC0402K  [C0402K]
C46  10uF  C-USC0805K  [C0805K]
C47  0.1uF  C-USC0402K  [C0402K]
C48  0.1uF  C-USC0402K  [C0402K]
C49  0.1uF  C-USC0402K  [C0402K]
C50  10uF  C-USC0805K  [C0805K]
J12  DNP  FTSH-105-01-F-DVFTSH-105-01-F-DV  [FTSH-105-01-F-DV]
R39  2.2k  R-US_R0402  [R0402]
R40  49.9  R-US_R0402  [R0402]
U8  LM4040D30_DBZ_3  [DBZ3]
Y2  16.00MHZ  CRYSTAL  [ABLS]

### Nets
+1V2_TM4C: C47.1 C49.1 C50.1 U7.87(B:VDDC) U7.115(B:VDDC)
+3V3: C35.1 C36.1 C37.1 C38.1 C40.1 C41.1 C42.1 C43.1 C44.1 C45.1 C46.1 J12.1 R39.1 R40.1 U7.7(B:VDD) U7.8(B:VDDA) U7.16(B:VDD) U7.26(B:VDD) U7.28(B:VDD) U7.39(B:VDD) U7.47(B:VDD) U7.51(C:VDD) U7.52(C:VDD) U7.68(B:VBAT) U7.69(B:VDD) U7.79(B:VDD) U7.90(B:VDD) U7.101(B:VDD) U7.113(B:VDD) U7.122(B:VDD) ; also sheet 2,3,5,6,7,8,9,10,11,12
GND: C34.2 C35.2 C36.2 C37.2 C38.2 C39.2 C40.2 C41.2 C42.2 C43.2 C44.2 C45.2 C46.2 C47.2 C48.2 C49.2 C50.2 J12.3 J12.5 J12.7 J12.9 U7.10(B:GNDA) U7.17(B:GND) U7.48(B:GND) U7.55(C:GND) U7.58(C:GND) U7.64(B:!WAKE) U7.66(B:XOSC0) U7.80(B:GND) U7.114(B:GND) U8.2(ANODE) ; also sheet 2,3,5,6,7,8,9,10,11,12,14
IRSTN: J12.10 R39.2 U7.70(B:!RST)
ITCK: J12.4 ; also sheet 12
ITDI: J12.8 ; also sheet 12
ITDO: J12.6 ; also sheet 12
ITMS: J12.2 ; also sheet 12
OSC0: C34.1 U7.88(B:OSC0) Y2.2
OSC1: C39.1 U7.89(B:OSC1) Y2.1
VREFA+: C48.1 R40.2 U7.9(B:VREFA+) U8.1(CATHODE)
Unconnected: U7.53(C:EN0RXIN) U7.54(C:EN0RXIP) U7.56(C:EN0TXON) U7.57(C:EN0TXOP) U7.59(C:RBIAS) U7.65(B:!HIB) U7.67(B:XOSC1) U8.3(NC)

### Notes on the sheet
- 3.0V ADC REFERENCE

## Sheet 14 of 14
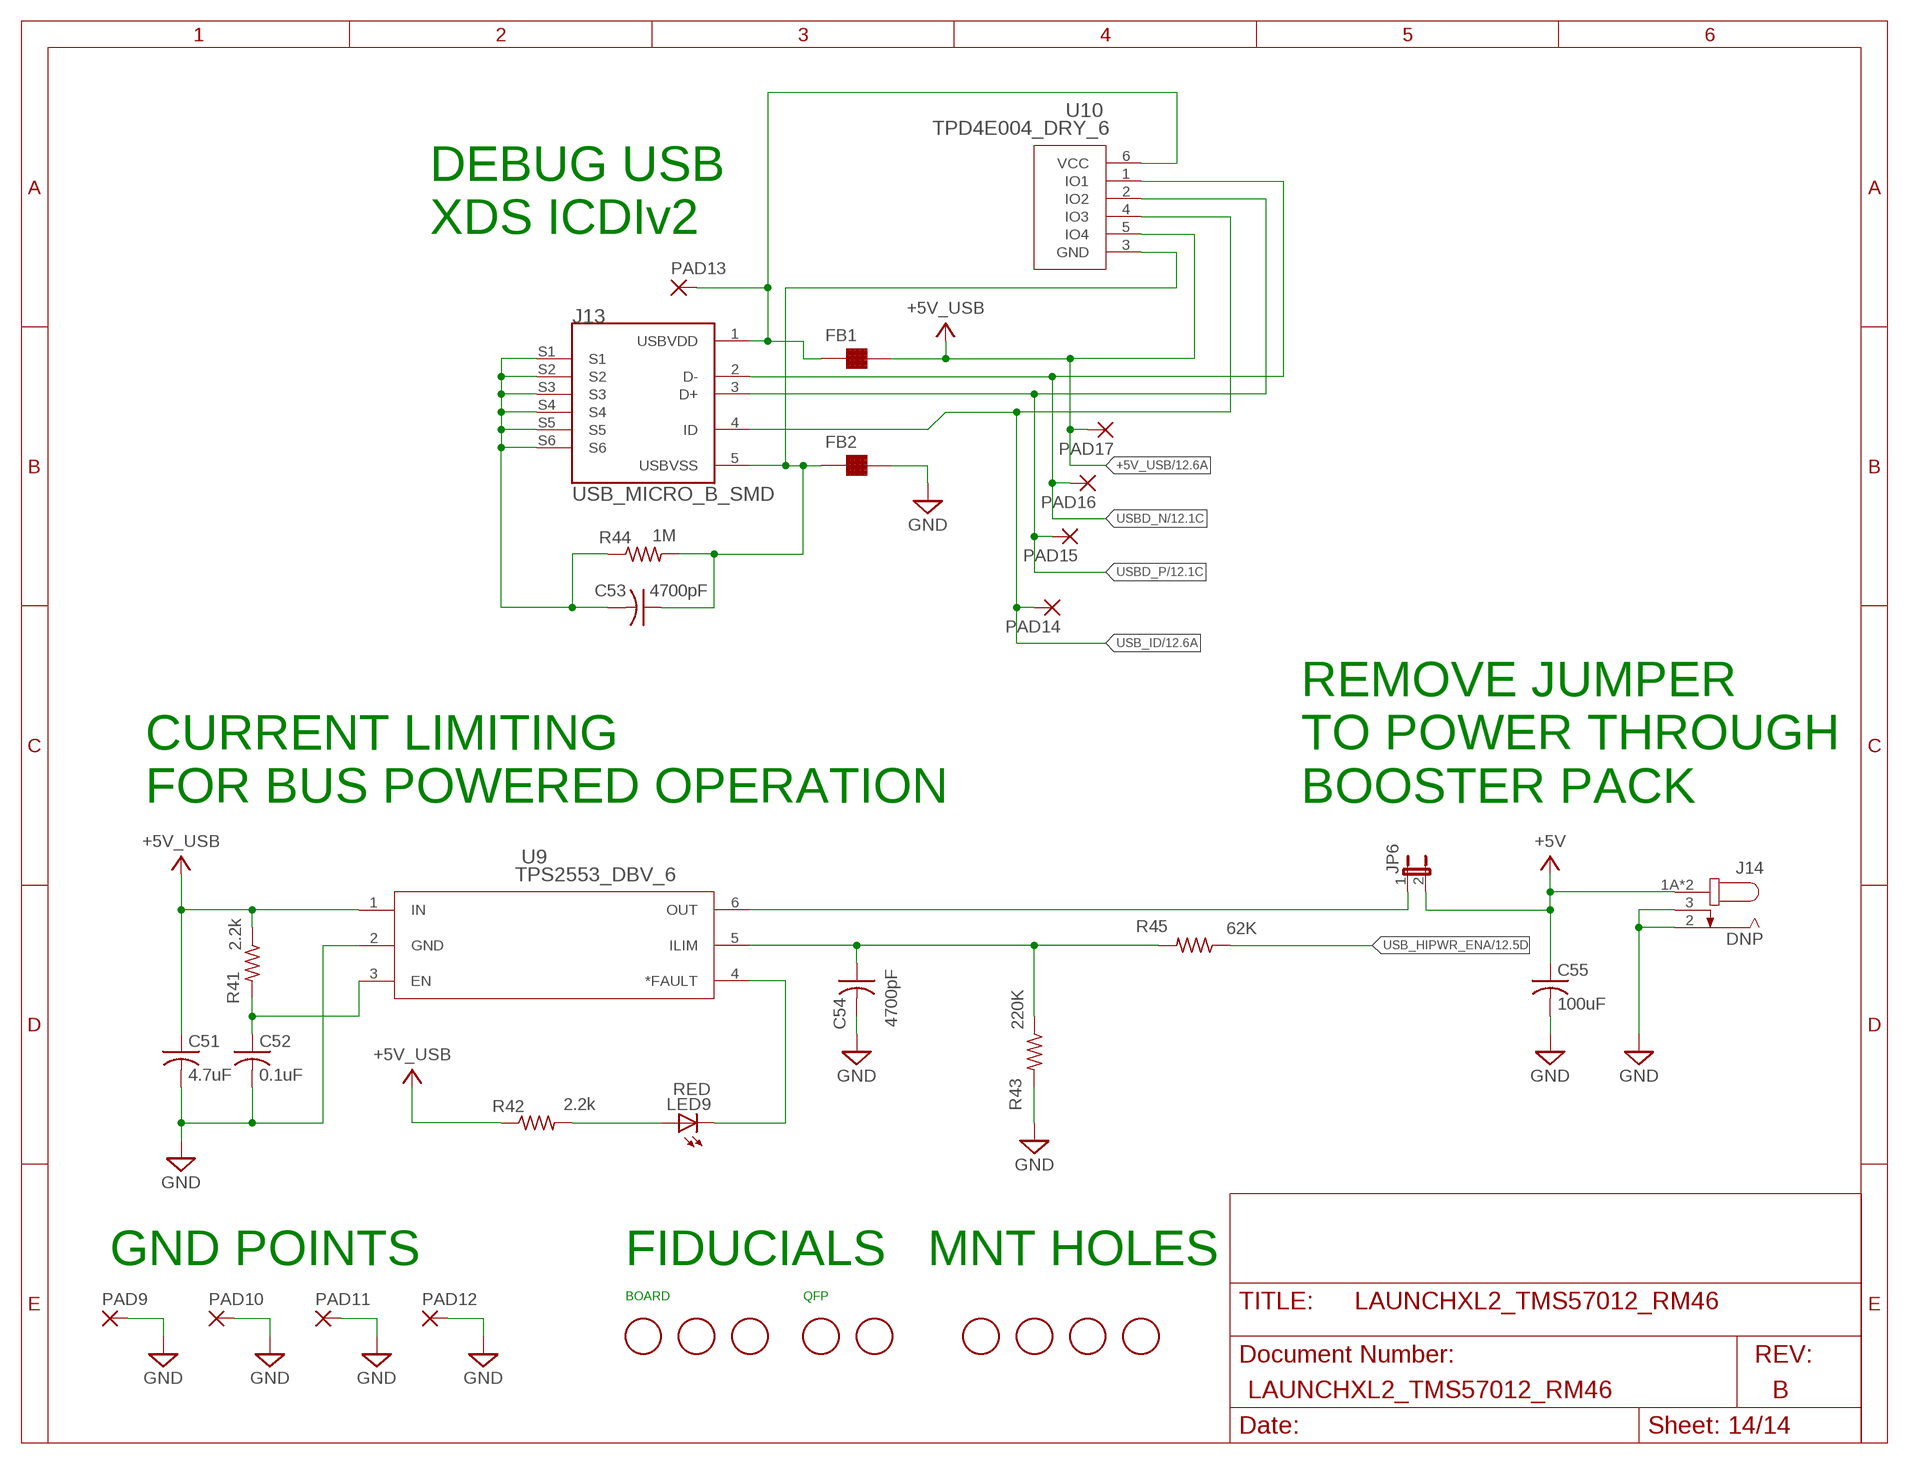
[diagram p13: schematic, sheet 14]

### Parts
C51  4.7uF  C-USC0603K  [C0603K]
C52  0.1uF  C-USC0402K  [C0402K]
C53  4700pF  C-USC0402K  [C0402K]
C54  4700pF  C-USC0402K  [C0402K]
C55  100uF  C-USC1206K  [C1206K]
FB1  23 OHM @ 100MHz  FERRITEBEAD2FB_MJ4516  [FB_MJ4516]
FB2  23 OHM @ 100MHz  FERRITEBEAD2FB_MJ4516  [FB_MJ4516]
FID1  DNP  FIDUCIAL  [FIDUCIAL_1MM]
FID2  DNP  FIDUCIAL  [FIDUCIAL_1MM]
FID3  DNP  FIDUCIAL  [FIDUCIAL_1MM]
FID4  DNP  FIDUCIAL  [FIDUCIAL_1MM]
FID5  DNP  FIDUCIAL  [FIDUCIAL_1MM]
J13  USB_MICRO_B_SMD  [USB_MICRO_B_SMD]
J14  DNP  JACK-PLUGCUI_PJ002BH  [CUI_PJ002BH]
JP6  SHUNT_ON  JP1E  [JP1]
LED9  RED  LEDCHIPLED_0603  [CHIPLED_0603]
MH1  DNP  MHMS_2_56  [MH_94_200]
MH2  DNP  MHMS_2_56  [MH_94_200]
MH3  DNP  MHMS_2_56  [MH_94_200]
MH4  DNP  MHMS_2_56  [MH_94_200]
PAD9  DNP  WIREPAD2,54/1,1  [2,54/1,1]
PAD10  DNP  WIREPAD2,54/1,1  [2,54/1,1]
PAD11  DNP  WIREPAD2,54/1,1  [2,54/1,1]
PAD12  DNP  WIREPAD2,54/1,1  [2,54/1,1]
PAD13  DNP  WIREPADSMD1,27-254  [SMD1,27-2,54]
PAD14  DNP  WIREPADSMD1,27-254  [SMD1,27-2,54]
PAD15  DNP  WIREPADSMD1,27-254  [SMD1,27-2,54]
PAD16  DNP  WIREPADSMD1,27-254  [SMD1,27-2,54]
PAD17  DNP  WIREPADSMD1,27-254  [SMD1,27-2,54]
R41  2.2k  R-US_R0402  [R0402]
R42  2.2k  R-US_R0402  [R0402]
R43  220K  R-US_R0402  [R0402]
R44  1M  R-US_R0402  [R0402]
R45  62K  R-US_R0402  [R0402]
U9  TPS2553_DBV_6  [DBV6]
U10  TPD4E004_DRY_6  [DRY6]

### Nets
5V_USB_LIMITED: JP6.1 U9.6(OUT)
+5V: C55.1 J14.1A J14.1B JP6.2 ; also sheet 2,7,8,9,11
+5V_USB: C51.1 FB1.2(B) PAD17.1(P) R41.1 R42.1 U9.1(IN) U10.5(IO4) ; also sheet 12
GND: C51.2 C52.2 C54.2 C55.2 FB2.2(B) J14.2 J14.3 PAD9.1(P) PAD10.1(P) PAD11.1(P) PAD12.1(P) R43.2 U9.2(GND) ; also sheet 2,3,5,6,7,8,9,10,11,12,13
N$7: C54.1 R43.1 R45.2 U9.5(ILIM)
N$8: LED9.A R42.2
N$23: C52.1 R41.2 U9.3(EN)
USB_HIPWR_ENA: R45.1 ; also sheet 12
USB_ID: J13.4(ID) PAD14.1(P) U10.4(IO3) ; also sheet 12
USB_PWRFAULT: LED9.C U9.4(*FAULT)
USB_SHIELD: C53.2 J13.S1 J13.S2 J13.S3 J13.S4 J13.S5 J13.S6 R44.1
USBD_N [USBD]: J13.2(D-) PAD16.1(P) U10.1(IO1) ; also sheet 12
USBD_P [USBD]: J13.3(D+) PAD15.1(P) U10.2(IO2) ; also sheet 12
USBVDD: FB1.1(A) J13.1(USBVDD) PAD13.1(P) U10.6(VCC)
USBVSS: C53.1 FB2.1(A) J13.5(USBVSS) R44.2 U10.3(GND)

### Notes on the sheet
- DEBUG USB
  XDS ICDIv2
- CURRENT LIMITING
  FOR BUS POWERED OPERATION
- REMOVE JUMPER
  TO POWER THROUGH
  BOOSTER PACK
- GND POINTS | FIDUCIALS | MNT HOLES
- BOARD | QFP

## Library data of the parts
+1V2 +1V2_EMU PAD9-PAD17 = lp_proto:WIREPAD: Wire PAD connect wire on PCB
C1 C2 C34 C39 = lp_proto:C-US: CAPACITOR, American symbol; MPN: CL05C330JB5NNNC; OC_DIGIKEY: 1276-1272-6-ND; SUPPLIER: Samsung; TOLERANCE: 5%; TYPE: NP0; VOLTAGE: 50V
C3 = lp_proto:C-US: CAPACITOR, American symbol; MPN: C0402C102K3RACTU; OC_DIGIKEY: 399-1031-6-ND; OC_NEWARK: 07J4431; SUPPLIER: KEMET; TOLERANCE: 10%; TYPE: X7R; VOLTAGE: 25V
C4 C8 C46 C50 = lp_proto:C-US: CAPACITOR, American symbol; MPN: C0805C106K8PACTU; OC_DIGIKEY: 399-4925-2-ND; OC_NEWARK: 57K6910; SUPPLIER: KEMET; TOLERANCE: 10%; TYPE: X5R; VOLTAGE: 10V
C5-C7 C9-C23 C29 C35-C38 C40-C45 C47-C49 C52 = lp_proto:C-US: CAPACITOR, American symbol; MPN: GRM155R61A104KA01D; OC_DIGIKEY: 490-1318-2-ND; OC_NEWARK: 18X5176; SUPPLIER: MURATA; TOLERANCE: 10%; TYPE: X5R; VOLTAGE: 10V
C24 C31 C53 C54 = lp_proto:C-US: CAPACITOR, American symbol; MPN: C0402C472K3RACTU; OC_DIGIKEY: 399-1035-6-ND; OC_NEWARK: 07J4449; SUPPLIER: KEMET; TOLERANCE: 10%; TYPE: X7R; VOLTAGE: 25
C25-C27 C30 C32 C33 = lp_proto:C-US: CAPACITOR, American symbol; MPN: CL21A226KQQNNNE; OC_DIGIKEY: 1276-2907-2-ND; SUPPLIER: SAMSUNG; TOLERANCE: 10%; TYPE: X5R; VOLTAGE: 6.3V
C28 = lp_proto:C-US: CAPACITOR, American symbol; MPN: GRM155R61A105KE15DC; OC_DIGIKEY: 490-3890-2-ND; SUPPLIER: MURATA; TOLERANCE: 10%; TYPE: X5R; VOLTAGE: 10V
C51 = lp_proto:C-US: CAPACITOR, American symbol; MPN: C0603C475M8PACTU; OC_DIGIKEY: 399-9100-6-ND; OC_NEWARK: 12N3601; SUPPLIER: KEMET; TOLERANCE: 20%; TYPE: X5R; VOLTAGE: 10V
C55 = lp_proto:C-US: CAPACITOR, American symbol; MPN: C1206C107M9PACTU; OC_DIGIKEY: 399-5620-2-ND; OC_NEWARK: 42M4769; SUPPLIER: KEMET; TOLERANCE: 20%; TYPE: X5R; VOLTAGE: 6.3V
FB1 FB2 = lp_proto:FERRITEBEAD2: A Ferrite Bead(Alternate symbol); MPN: FBMJ4516HL230NT; OC_DIGIKEY: FBMJ4516HL230NT-ND; SUPPLIER: TAIYO YUDEN
FID1-FID5 = lp_proto:FIDUCIAL: For use by pick and place machines to calibrate the vision/machine, 1mm
J1 = lp_proto:PINHD-2X10: PIN HEADER; MPN: FTR-110-51-S-D-06; OC_DIGIKEY: FTR-110-51-S-D-06-ND; SUPPLIER: SAMTEC
J2 J4 J6 J8 = lp_proto:PINHD-1X10: PIN HEADER; MPN: SSQ-110-04-F-D; OC_DIGIKEY: SAM1204-10-ND; SUPPLIER: SAMTEC
J3 = lp_proto:PINHD-1X10: PIN HEADER; MPN: N/A - Combined with J2
J5 = lp_proto:PINHD-1X10: PIN HEADER; MPN: N/A - Combined with J4
J7 = lp_proto:PINHD-1X10: PIN HEADER; MPN: N/A - Combined with J6
J9 = lp_proto:PINHD-1X10: PIN HEADER; MPN: N/A - Combined with J8
J10 = lp_proto:PINHD-1X50; MPN: HTSW-150-07-G-S-ND; OC_DIGIKEY: HTSW-150-07-G-S; SUPPLIER: SAMTEC
J11 = lp_proto:PINHD-1X50; MPN: HTSW-150-07-G-S; OC_DIGIKEY: HTSW-150-07-G-S-ND; SUPPLIER: SAMTEC
J12 = lp_proto:FTSH-105-01-F-DV; MPN: FTSH-105-01-F-DV; OC_DIGIKEY: FTSH-105-01-F-DV-ND; SUPPLIER: SAMTEC
J13 = champ_lp_proto:USB_MICRO_B_SMD; MPN: 10104110-0001LF; OC_DIGIKEY: 609-4052-1-ND; SUPPLIER: FCI
J14 = lp_proto:JACK-PLUG: DC POWER JACK Power Jack, DC, Right Angle, Through Hole, Rated 5A at 16VDC, PC Terminals Distributor: Farnell (www.Farnell.de) Drawing: 84N1161.pdf / 84N1162.pdf Manufacturer: SPC Technology (www.spctechnology.com) Type: SPC4077 / SPC 4078; MPN: PJ-002BH-SMT-TR; OC_DIGIKEY: CP-002BHPJTR-ND; SUPPLIER: CUI
JP1-JP6 = lp_proto:JP1E: JUMPER; MPN: HTSW-102-07-G-S; OC_DIGIKEY: SAM8736-ND; SUPPLIER: SAMTEC
L1 L2 = lp_proto:L-US: INDUCTOR, American symbol; CURRENT: 3.1A; MPN: 252012CDMCDS-1R0MC; OC_DIGIKEY: 308-2342-2-ND; SUPPLIER: SUMIDA AMERICA
LED1 LED9 = lp_proto:LED: LED; COLOR: RED; MPN: LTST-C191KRKT; OC_DIGIKEY: 160-1447-2-ND; SUPPLIER: LITE ON
LED2-LED4 LED6-LED8 = lp_proto:LED: LED; COLOR: GRN; MPN: LTST-C191KGKT; OC_DIGIKEY: 160-1446-2-ND; SUPPLIER: LITE ON
MH1-MH4 = champ_lp_proto:MH
Q1 = champ_lp_proto:TEMT6000; MPN: TEMT6000X01; OC_DIGIKEY: 751-1055-1-ND; SUPPLIER: VISHAY
R1-R3 = lp_proto:R-US_: RESISTOR, American symbol; MPN: RMCF0402ZT0R00; OC_DIGIKEY: RMCF0402ZT0R00TR-ND; OC_NEWARK: 62X8436; SUPPLIER: VISHAY/STACKPOLE; TOLERANCE: 1%
R4 = lp_proto:R-US_: RESISTOR, American symbol
R5 R7-R11 R13 R15-R17 R22 R27 R32 R33 R39 R41 R42 = lp_proto:R-US_: RESISTOR, American symbol; MPN: RMCF0402JT2K20; OC_DIGIKEY: RMCF0402JT2K20TR-ND; OC_NEWARK: 67K8915; SUPPLIER: VISHAY/STACKPOLE; TOLERANCE: 1%
R6 R19 R26 = lp_proto:R-US_: RESISTOR, American symbol; MPN: RMCF0402FT10K0; OC_DIGIKEY: RMCF0402FT10K0TR-ND; OC_NEWARK: 19K7996; SUPPLIER: VISHAY/STACKPOLE; TOLERANCE: 1%
R12 = lp_proto:R-US_: RESISTOR, American symbol; MPN: RMCF0402JT33R0; OC_DIGIKEY: RMCF0402JT33R0TR-ND; OC_NEWARK: 19K8702; SUPPLIER: VISHAY/STACKPOLE; TOLERANCE: 5%
R14 R25 = lp_proto:R-US_: RESISTOR, American symbol; MPN: RMCF0402FT5K76; OC_DIGIKEY: RMCF0402FT5K76TR-ND; SUPPLIER: STACKPOLE; TOLERANCE: 1%
R18 R28 = lp_proto:R-US_: RESISTOR, American symbol; MPN: RMCF0402FT31K6; OC_DIGIKEY: RMCF0402FT31K6TR-ND; OC_NEWARK: 52K6966; SUPPLIER: VISHAY/STACKPOLE; TOLERANCE: 1%
R21 = lp_proto:R-US_: RESISTOR, American symbol; MPN: RMCF0402FT4R99; OC_DIGIKEY: RMCF0402FT4R99TR-ND; SUPPLIER: STACKPOLE; TOLERANCE: 1%
R29 = lp_proto:R-US_: RESISTOR, American symbol; MPN: PF1206FRF070R01L; OC_DIGIKEY: 311-0.01AJTR-ND; SUPPLIER: YAGEO; TOLERANCE: 1%
R30 R31 = lp_proto:R-US_: RESISTOR, American symbol; MPN: RMCF0402FT330K; OC_DIGIKEY: RMCF0402FT330KTR-ND; SUPPLIER: STACKPOLE; TOLERANCE: 1%
R34 R35 R43 = lp_proto:R-US_: RESISTOR, American symbol; MPN: CRCW0402220KFKED; OC_DIGIKEY: 541-220KLTR-ND; OC_NEWARK: 43C3674; SUPPLIER: VISHAY/STACKPOLE; TOLERANCE: 1%
R40 = lp_proto:R-US_: RESISTOR, American symbol; MPN: RMCF0402FT49R9; OC_DIGIKEY: RMCF0402FT49R9TR-ND; OC_NEWARK: 52K7115; SUPPLIER: VISHAY/STACKPOLE; TOLERANCE: 1%
R44 = lp_proto:R-US_: RESISTOR, American symbol; MPN: RMCF0402FT1M00; OC_DIGIKEY: RMCF0402FT1M00DKR-ND; SUPPLIER: STACKPOLE; TOLERANCE: 1%
R45 = lp_proto:R-US_: RESISTOR, American symbol; MPN: CRCW040262K0FKED; OC_DIGIKEY: 541-62.0KLTR-ND; OC_NEWARK: 89M6683; SUPPLIER: VISHAY/STACKPOLE; TOLERANCE: 1%
S1-S4 = lp_proto:TACT6MM_NO_MOM; MPN: PTS645SM43SMTR92 LFS; OC_DIGIKEY: CKN9112TR-ND; SUPPLIER: C&K Components; TYPE: SPST-NO-MOM
U1 = champ_lp_proto:RM46L850_PGE_144; MANUFACTURER_PART_NUMBER: rm46l850_pge_144; MPN: RM46L852PGET; OC_DIGIKEY: 296-37040-ND; SUPPLIER: TI; VENDOR: TEXAS INSTRUMENTS
U2 = lp_proto:TPS3106K33_DBV_6; DATASHEETURL: http://www.ti.com/lit/gpn/TPS3106K33; DESCRIPTION: Ultra Low-Supply Current/Supply-Voltage Supervisory Circuits; FAMILY_NAME: SUPERVISOR AND RESET IC; GENERIC_PART_NUMBER: TPS3106K33; INDUSTRY_STD_PKG_TYPE: SOT-23; MANUFACTURER: Texas Instruments; MANUFACTURER_PART_NUMBER: tps3106k33_dbv_6; MPN: TPS3106K33DBVR; OC_DIGIKEY: 296-13399-2-ND; OC_NEWARK: 77C0262; PACKAGE_DESIGNATOR: DBV; PIN_COUNT: 6; SUPPLIER: TI; VENDOR: Texas Instruments
U5 = lp_proto:LM26420_PWP_20; FREQ: 2.2MHz; MANUFACTURER_PART_NUMBER: LM26420XMH/NOPB; MPN: LM26420XMH/NOPB; OC_DIGIKEY: LM26420XMHX/NOPB-ND; OC_NEWARK: 14R4583; SUPPLIER: TI; VENDOR: Texas Instruments
U6 = lp_proto:INA210_DCK_6; DATASHEETURL: http://www.ti.com/lit/gpn/INA210; DESCRIPTION: Voltage Output, High/Low-Side Measurement, Bi-Directional Zero-Drift Series Current Shunt Monitor; FAMILY_NAME: CURRENT SHUNT MONITOR; GENERIC_PART_NUMBER: INA210; INDUSTRY_STD_PKG_TYPE: SC70; MANUFACTURER: Texas Instruments; MANUFACTURER_PART_NUMBER: ina210_dck_6; MPN: INA210BIDCKR; OC_DIGIKEY: INA210BIDCKR-ND; PACKAGE_DESIGNATOR: DCK; PIN_COUNT: 6; SUPPLIER: TI; VENDOR: Texas Instruments
U7 = lp_proto:TM4C129ENCPDT; MANUFACTURER_PART_NUMBER: TM4C129ENCPDT; MPN: TM4C129ENCPDTI3; OC_DIGIKEY: 296-37940-ND; SUPPLIER: TI; VENDOR: Texas Instruments
U8 = champ_lp_proto:LM4040D30_DBZ_3; DATASHEETURL: http://www.ti.com/lit/gpn/LM4040D30; DESCRIPTION: 3-V Precision Micropower Shunt Voltage Reference, 1% accuracy; FAMILY_NAME: SHUNT VOLTAGE REFERENCE; GENERIC_PART_NUMBER: LM4040D30; INDUSTRY_STD_PKG_TYPE: SOT-23; MANUFACTURER: Texas Instruments; MANUFACTURER_PART_NUMBER: lm4040d30_dbz_3; OC_DIGIKEY: 296-19437-2-ND; PACKAGE_DESIGNATOR: DBZ; PIN_COUNT: 3; VENDOR: Texas Instruments
U9 = lp_proto:TPS2553_DBV_6; DATASHEETURL: http://www.ti.com/lit/gpn/TPS2553; DESCRIPTION: Adjustable, Active High, Constant-Current, Current-Limited Power-Distribution Switch; FAMILY_NAME: USB POWER SWITCH; GENERIC_PART_NUMBER: TPS2553; INDUSTRY_STD_PKG_TYPE: SOT-23; MANUFACTURER: Texas Instruments; MANUFACTURER_PART_NUMBER: tps2553_dbv_6; MPN: TPS2553DBVR; OC_DIGIKEY: 296-32464-2-ND; PACKAGE_DESIGNATOR: DBV; PIN_COUNT: 6; SUPPLIER: TI; VENDOR: Texas Instruments
U10 = lp_proto:TPD4E004_DRY_6; DATASHEETURL: http://www.ti.com/lit/gpn/TPD4E004; DESCRIPTION: 4-Channel ESD Protection Array for High-Speed Data Interfaces; FAMILY_NAME: ESD Solution; GENERIC_PART_NUMBER: TPD4E004; INDUSTRY_STD_PKG_TYPE: SON; MANUFACTURER: Texas Instruments; MANUFACTURER_PART_NUMBER: tpd4e004_dry_6; MPN: TPD4E004DRYR; OC_DIGIKEY: 296-23618-2-ND; PACKAGE_DESIGNATOR: DRY; PIN_COUNT: 6; SUPPLIER: TI; VENDOR: Texas Instruments
Y1 Y2 = lp_proto:CRYSTAL: CRYSTAL; MPN: ABLS-16.000MHZ-B4-T; OC_DIGIKEY: 535-10226-2-ND; SUPPLIER: ABRACON

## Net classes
0 default: width 0.152 mm, drill 0.381 mm
1 USBD: width 0.356 mm, drill 0.381 mm, clearance 0.152 mm to class 0, clearance 0.152 mm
